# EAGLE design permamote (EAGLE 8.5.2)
AUTHOR: NEAL JACKSON; REV: A; TITLE: MOTE

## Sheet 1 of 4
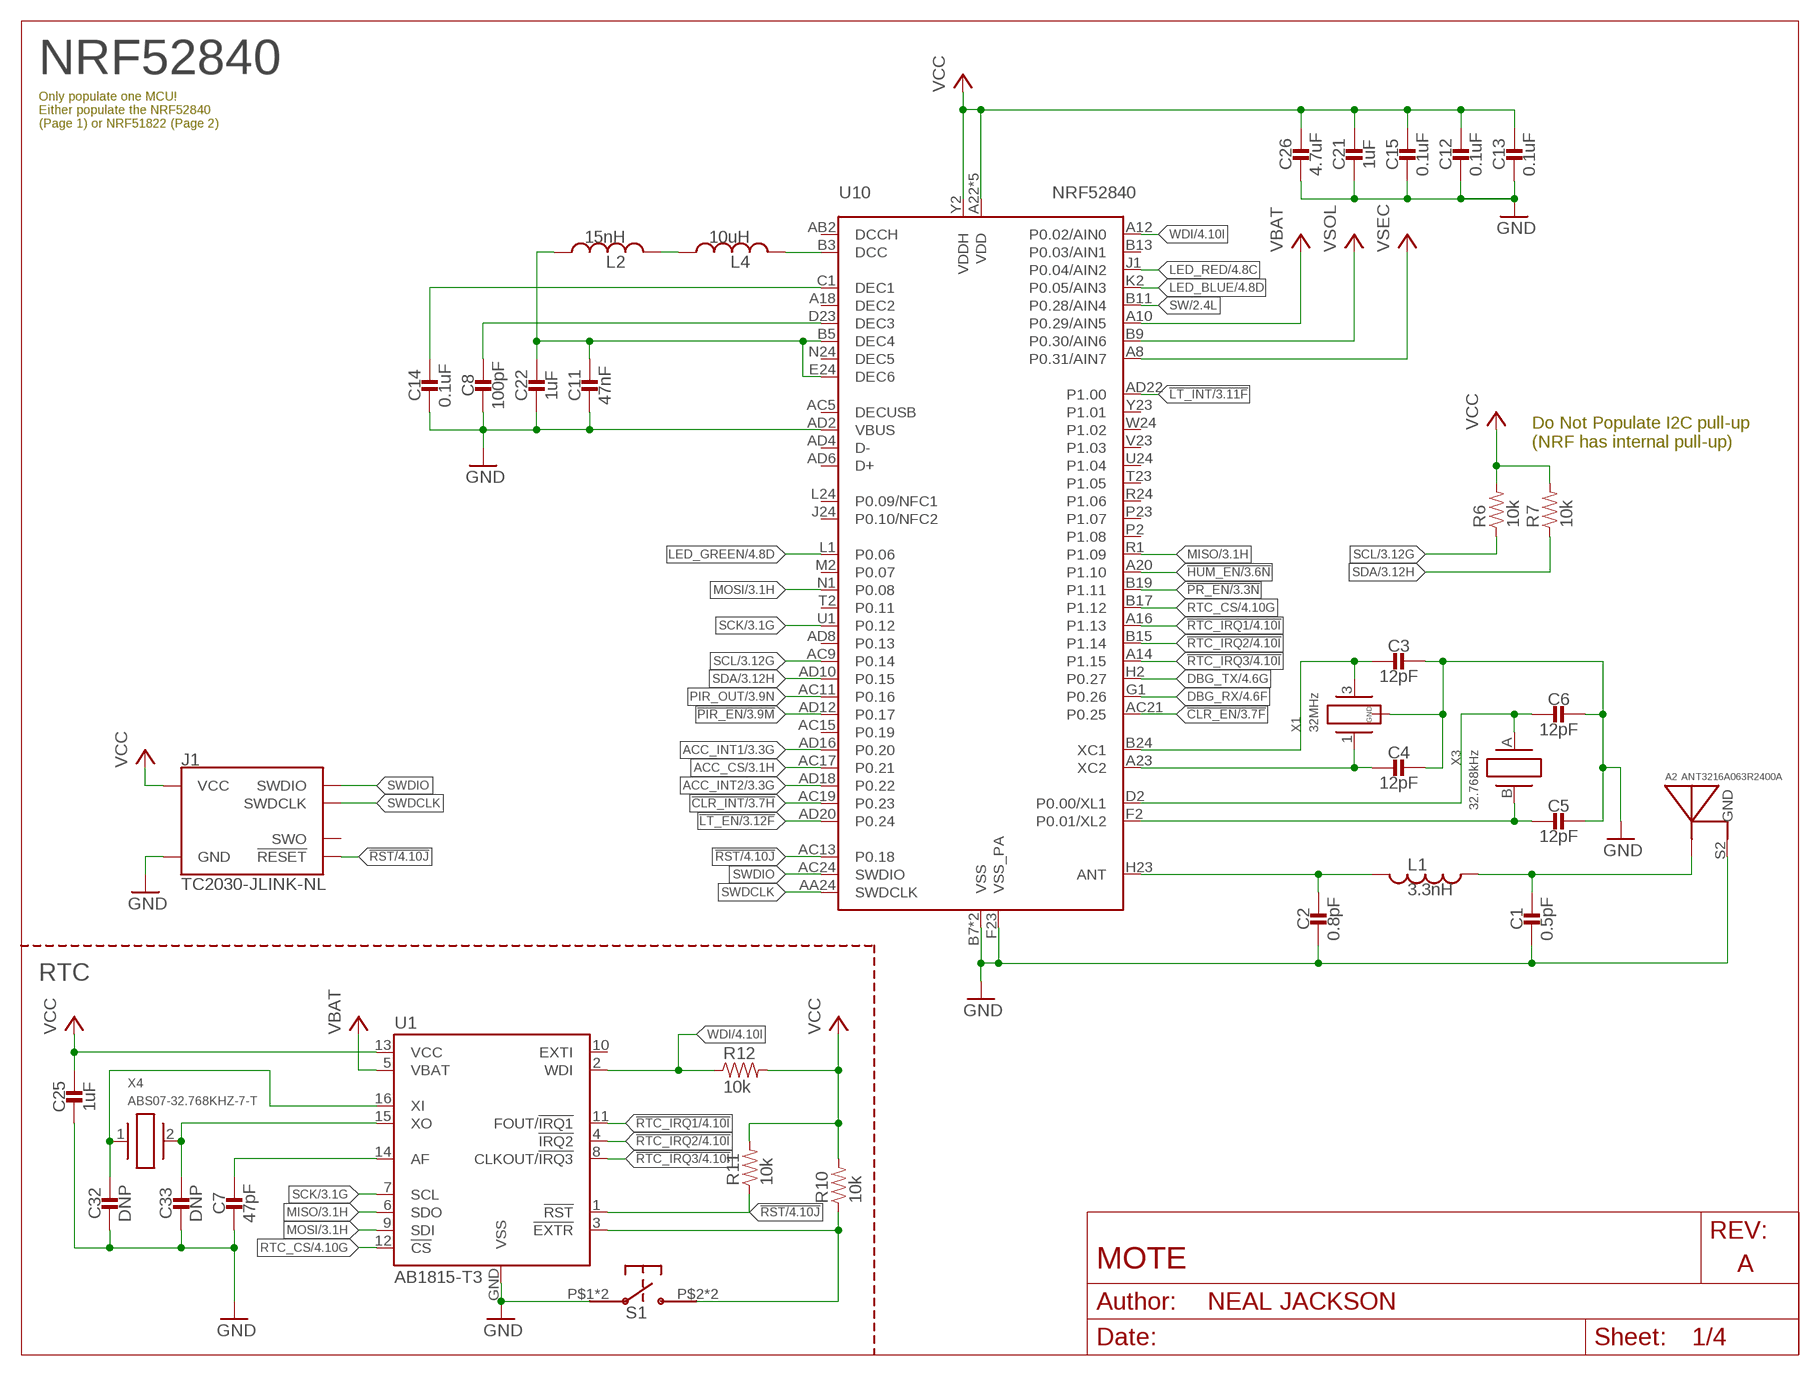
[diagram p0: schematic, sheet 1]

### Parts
A2  ANT3216A063R2400A  [ANT3216A063R2400A]
C1  0.5pF  CAPACITOR0402_CAP  [0402_CAP]
C2  0.8pF  CAPACITOR0402_CAP  [0402_CAP]
C3  12pF  CAPACITOR0402_CAP  [0402_CAP]
C4  12pF  CAPACITOR0402_CAP  [0402_CAP]
C5  12pF  CAPACITOR0402_CAP  [0402_CAP]
C6  12pF  CAPACITOR0402_CAP  [0402_CAP]
C7  47pF  CAPACITOR0402_CAP  [0402_CAP]
C8  100pF  CAPACITOR0402_CAP  [0402_CAP]
C11  47nF  CAPACITOR0402_CAP  [0402_CAP]
C12  0.1uF  CAPACITOR0402_CAP  [0402_CAP]
C13  0.1uF  CAPACITOR0402_CAP  [0402_CAP]
C14  0.1uF  CAPACITOR0402_CAP  [0402_CAP]
C15  0.1uF  CAPACITOR0402_CAP  [0402_CAP]
C21  1uF  CAPACITOR0402_CAP  [0402_CAP]
C22  1uF  CAPACITOR0402_CAP  [0402_CAP]
C25  1uF  CAPACITOR0402_CAP  [0402_CAP]
C26  4.7uF  CAPACITOR0402_CAP  [0402_CAP]
C32  DNP  CAPACITOR0402_CAP  [0402_CAP]
C33  DNP  CAPACITOR0402_CAP  [0402_CAP]
J1  TC2030-JLINK-NL  [TC2030-IDC-NL]
L1  3.3nH  INDUCTOR0402  [0402_CAP]
L2  15nH  INDUCTOR0402  [0402_CAP]
L4  10uH  INDUCTOR0603  [0603_CAP]
R6  10k  RESISTOR0402_RES  [0402_RES]
R7  10k  RESISTOR0402_RES  [0402_RES]
R10  10k  RESISTOR0402_RES  [0402_RES]
R11  10k  RESISTOR0402_RES  [0402_RES]
R12  10k  RESISTOR0402_RES  [0402_RES]
S1  EVQP2  [EVQP2]
U1  AB1815-T3  [QFN-16-3MM]
U10  NRF52840  [AQFN73]
X1  32MHz  7V-32.000MAHV-T  [TXC-7V]
X3  32.768kHz  ABS05-32.768KHZ-9-T  [ABS05]
X4  ABS07-32.768KHZ-7-T  [2-SMD]

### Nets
!CLR_EN: U10.AC21(P0.25) ; also sheet 3,4
!CLR_INT: U10.AC19(P0.23) ; also sheet 3,4
!HUM_EN: U10.A20(P1.10) ; also sheet 3,4
!LT_EN: U10.AD20(P0.24) ; also sheet 3,4
!LT_INT: U10.AD22(P1.00) ; also sheet 3,4
!PIR_EN: U10.AD12(P0.17) ; also sheet 3,4
!PR_EN: U10.B19(P1.11) ; also sheet 3,4
!RST: J1.3(!RESET) R11.1 U1.1(!RST) U10.AC13(P0.18) ; also sheet 4
!RTC_EXTR: R10.1 S1.P$2 S1.P$4 U1.3(!EXTR)
!RTC_IRQ1: U1.11(FOUT/!IRQ1) U10.A16(P1.13) ; also sheet 4
!RTC_IRQ2: U1.4(!IRQ2) U10.B15(P1.14) ; also sheet 4
!RTC_IRQ3: U1.8(CLKOUT/!IRQ3) U10.A14(P1.15) ; also sheet 4
ACC_CS: U10.AC17(P0.21) ; also sheet 3,4
ACC_INT1: U10.AD16(P0.20) ; also sheet 3,4
ACC_INT2: U10.AD18(P0.22) ; also sheet 3,4
DBG_RX: U10.G1(P0.26) ; also sheet 4
DBG_TX: U10.H2(P0.27) ; also sheet 4
GND: A2.S2(GND) C1.2 C2.2 C3.1 C4.1 C5.1 C6.1 C7.2 C8.2 C11.2 C12.2 C13.2 C14.2 C15.2 C21.2 C22.2 C25.2 C26.2 C32.2 C33.2 J1.5(GND) S1.P$1 S1.P$3 U1.GND(VSS) U10.AD2(VBUS) U10.B7(VSS) U10.F23(VSS_PA) U10.GND(VSS) X1.2(GND) X1.4(GND) ; also sheet 2,3,4
LED_BLUE: U10.K2(P0.05/AIN3) ; also sheet 4
LED_GREEN: U10.L1(P0.06) ; also sheet 4
LED_RED: U10.J1(P0.04/AIN2) ; also sheet 4
MISO: U1.6(SDO) U10.R1(P1.09) ; also sheet 3,4
MOSI: U1.9(SDI) U10.N1(P0.08) ; also sheet 3,4
N$2: C14.1 U10.C1(DEC1)
N$3: C11.1 C22.1 L2.1 U10.B5(DEC4) U10.E24(DEC6)
N$4: C8.1 U10.D23(DEC3)
N$5: C2.1 L1.2 U10.H23(ANT)
N$6: A2.S1(ANTENNA) C1.1 L1.1
N$8: C3.2 U10.B24(XC1) X1.3
N$9: C4.2 U10.A23(XC2) X1.1
N$25: C7.1 U1.14(AF)
N$26: C32.1 U1.16(XI) X4.1
N$27: C33.1 U1.15(XO) X4.2
N$44: L4.2 U10.B3(DCC)
N$49: L2.2 L4.1
PIR_OUT: U10.AC11(P0.16) ; also sheet 3,4
RTC_CS: U1.12(!CS) U10.B17(P1.12) ; also sheet 4
SCK: U1.7(SCL) U10.U1(P0.12) ; also sheet 3,4
SCL: R6.1 U10.AC9(P0.14) ; also sheet 3,4
SDA: R7.1 U10.AD10(P0.15) ; also sheet 3,4
SW: U10.B11(P0.28/AIN4) ; also sheet 2,4
SWDCLK: J1.4(SWDCLK) U10.AA24(SWDCLK)
SWDIO: J1.2(SWDIO) U10.AC24(SWDIO)
VBAT: U1.5(VBAT) U10.A10(P0.29/AIN5) ; also sheet 2
VCC: C12.1 C13.1 C15.1 C21.1 C25.1 C26.1 J1.1(VCC) R6.2 R7.2 R10.2 R11.2 R12.2 U1.13(VCC) U10.A22(VDD) U10.AD14(VDD) U10.AD23(VDD) U10.B1(VDD) U10.W1(VDD) U10.Y2(VDDH) ; also sheet 2,3,4
VSEC: U10.A8(P0.31/AIN7) ; also sheet 2,4
VSOL: U10.B9(P0.30/AIN6) ; also sheet 2,4
WDI: R12.1 U1.2(WDI) U10.A12(P0.02/AIN0) ; also sheet 4
XL1: C6.2 U10.D2(P0.00/XL1) X3.A
XL2: C5.2 U10.F2(P0.01/XL2) X3.B
Unconnected: J1.6(SWO) U1.10(EXTI) U10.A18(DEC2) U10.AB2(DCCH) U10.AC5(DECUSB) U10.AC15(P0.19) U10.AD4(D-) U10.AD6(D+) U10.AD8(P0.13) U10.B13(P0.03/AIN1) U10.J24(P0.10/NFC2) U10.L24(P0.09/NFC1) U10.M2(P0.07) U10.N24(DEC5) U10.P2(P1.08) U10.P23(P1.07) U10.R24(P1.06) U10.T2(P0.11) U10.T23(P1.05) U10.U24(P1.04) U10.V23(P1.03) U10.W24(P1.02) U10.Y23(P1.01)

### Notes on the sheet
- NRF52840
- Only populate one MCU!
  Either populate the NRF52840
  (Page 1) or NRF51822 (Page 2)
- Do Not Populate I2C pull-up
  (NRF has internal pull-up)
- RTC

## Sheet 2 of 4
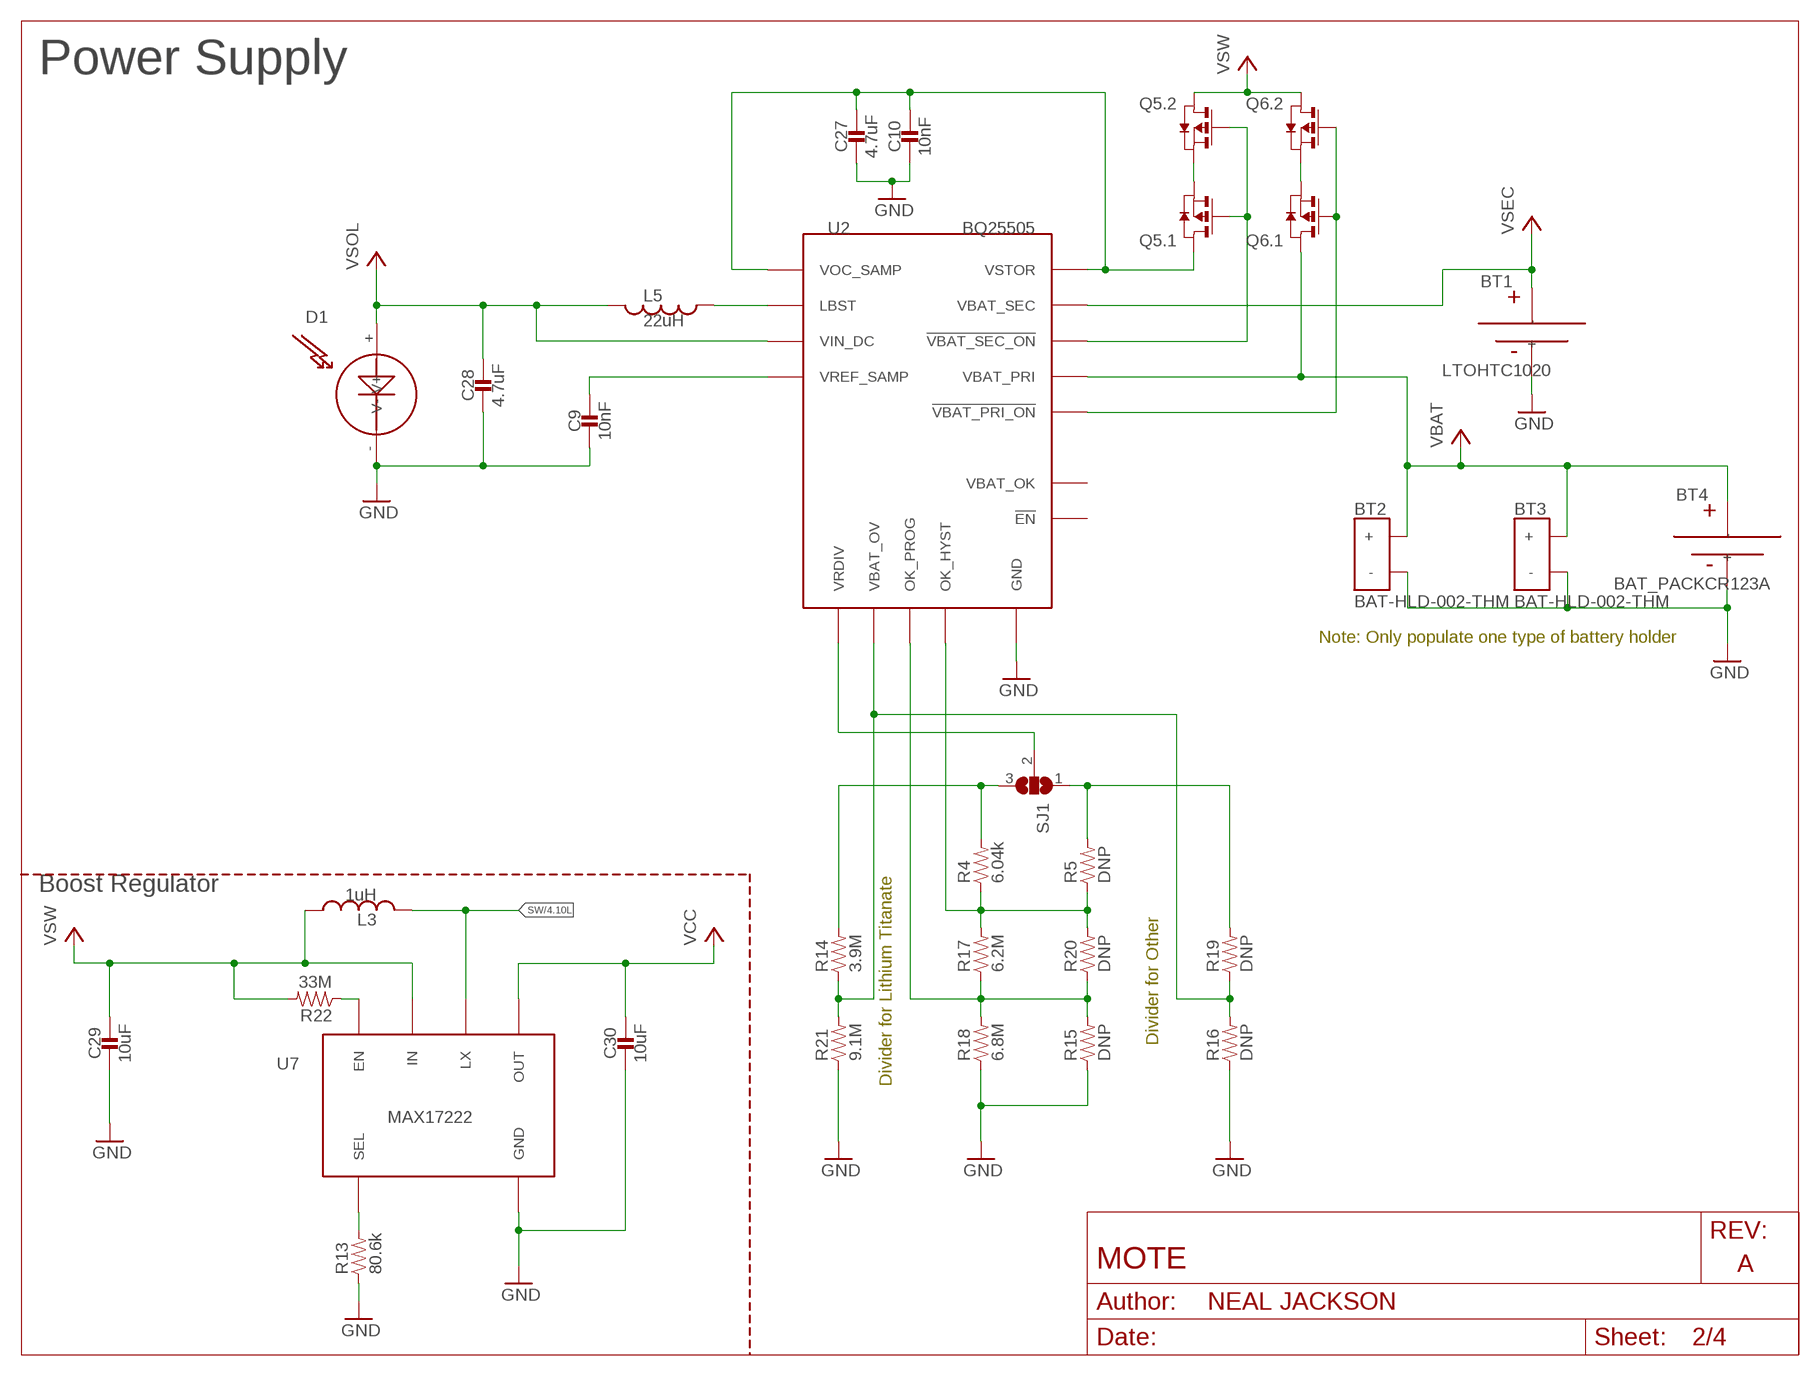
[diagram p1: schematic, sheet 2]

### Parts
BT1  LTOHTC1020  [1020]
BT2  BAT-HLD-002-THM  [BAT-HLD-002-THM]
BT3  BAT-HLD-002-THM  [BAT-HLD-002-THM]
BT4  BAT_PACKCR123A  [BH123A]
C9  10nF  CAPACITOR0402_CAP  [0402_CAP]
C10  10nF  CAPACITOR0402_CAP  [0402_CAP]
C27  4.7uF  CAPACITOR0402_CAP  [0402_CAP]
C28  4.7uF  CAPACITOR0402_CAP  [0402_CAP]
C29  10uF  CAPACITOR0603_CAP  [0603_CAP]
C30  10uF  CAPACITOR0603_CAP  [0603_CAP]
D1  SOLARCELLHOLES  [SOLAR_HOLES]
L3  1uH  INDUCTORIHL  [IHL-1212BZ-11]
L5  22uH  INDUCTOR74437324220  [74437324220]
Q5  PMDXB950UPEL  [XDFN-6]
Q6  PMDXB950UPEL  [XDFN-6]
R4  6.04k  RESISTOR0402_RES  [0402_RES]
R5  DNP  RESISTOR0402_RES  [0402_RES]
R13  80.6k  RESISTOR0603_RES  [0603-RES]
R14  3.9M  RESISTOR0402_RES  [0402_RES]
R15  DNP  RESISTOR0402_RES  [0402_RES]
R16  DNP  RESISTOR0402_RES  [0402_RES]
R17  6.2M  RESISTOR0402_RES  [0402_RES]
R18  6.8M  RESISTOR0402_RES  [0402_RES]
R19  DNP  RESISTOR0402_RES  [0402_RES]
R20  DNP  RESISTOR0402_RES  [0402_RES]
R21  9.1M  RESISTOR0402_RES  [0402_RES]
R22  33M  RESISTOR0603_RES  [0603-RES]
SJ1  SJ2W  [SJ_2]
U2  BQ25505  [S-PVQFN-N20-RGR]
U7  MAX17222  [UDFN-6-MAXIM]

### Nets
!VBAT_PRI_ON: Q6.2(.1:G) Q6.5(.2:G) U2.10(!VBAT_PRI_ON)
!VBAT_SEC_ON: Q5.2(.1:G) Q5.5(.2:G) U2.9(!VBAT_SEC_ON)
GND: BT1.- BT2.GND(-) BT3.GND(-) BT4.- C9.2 C10.2 C27.2 C28.2 C29.2 C30.2 D1.-(V-) R13.1 R15.1 R16.1 R18.1 R21.1 U2.1(GND) U2.6(GND) U2.15(GND) U2.16(GND) U2.17(GND) U2.PAD(GND) U7.3(GND) ; also sheet 1,3,4
LBST: L5.P$1 U2.20(LBST)
N$1: R4.2 R14.2 SJ1.3
N$12: R13.2 U7.4(SEL)
N$14: R22.1 U7.6(EN)
N$16: R5.2 R19.2 SJ1.1
N$18: R14.1 R16.2 R19.1 R21.2 U2.7(VBAT_OV)
N$32: SJ1.2 U2.8(VRDIV)
N$45: Q5.1(.1:S) Q5.4(.2:S)
N$53: Q6.1(.1:S) Q6.4(.2:S)
N$57: R15.2 R17.1 R18.2 R20.1 U2.12(OK_PROG)
N$58: R4.1 R5.1 R17.2 R20.2 U2.11(OK_HYST)
SW: L3.P$2 U7.2(LX) ; also sheet 1,4
VBAT: BT2.POS1(+) BT2.POS2(+) BT2.POS3(+) BT2.POS4(+) BT3.POS1(+) BT3.POS2(+) BT3.POS3(+) BT3.POS4(+) BT4.+ Q6.6(.1:D) U2.14(VBAT_PRI) ; also sheet 1
VCC: C30.1 U7.1(OUT) ; also sheet 1,3,4
VOC_SAMP_VSTOR: C10.1 C27.1 Q5.6(.1:D) U2.3(VOC_SAMP) U2.19(VSTOR)
VREF_SAMP: C9.1 U2.4(VREF_SAMP)
VSEC: BT1.+ U2.18(VBAT_SEC) ; also sheet 1,4
VSOL: C28.1 D1.+(V+) L5.P$2 U2.2(VIN_DC) ; also sheet 1,4
VSW: C29.1 L3.P$1 Q5.3(.2:D) Q6.3(.2:D) R22.2 U7.5(IN)
Unconnected: U2.5(!EN) U2.13(VBAT_OK)

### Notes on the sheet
- Power Supply
- Note: Only populate one type of battery holder
- Boost Regulator
- Divider for Lithium Titanate | Divider for Other

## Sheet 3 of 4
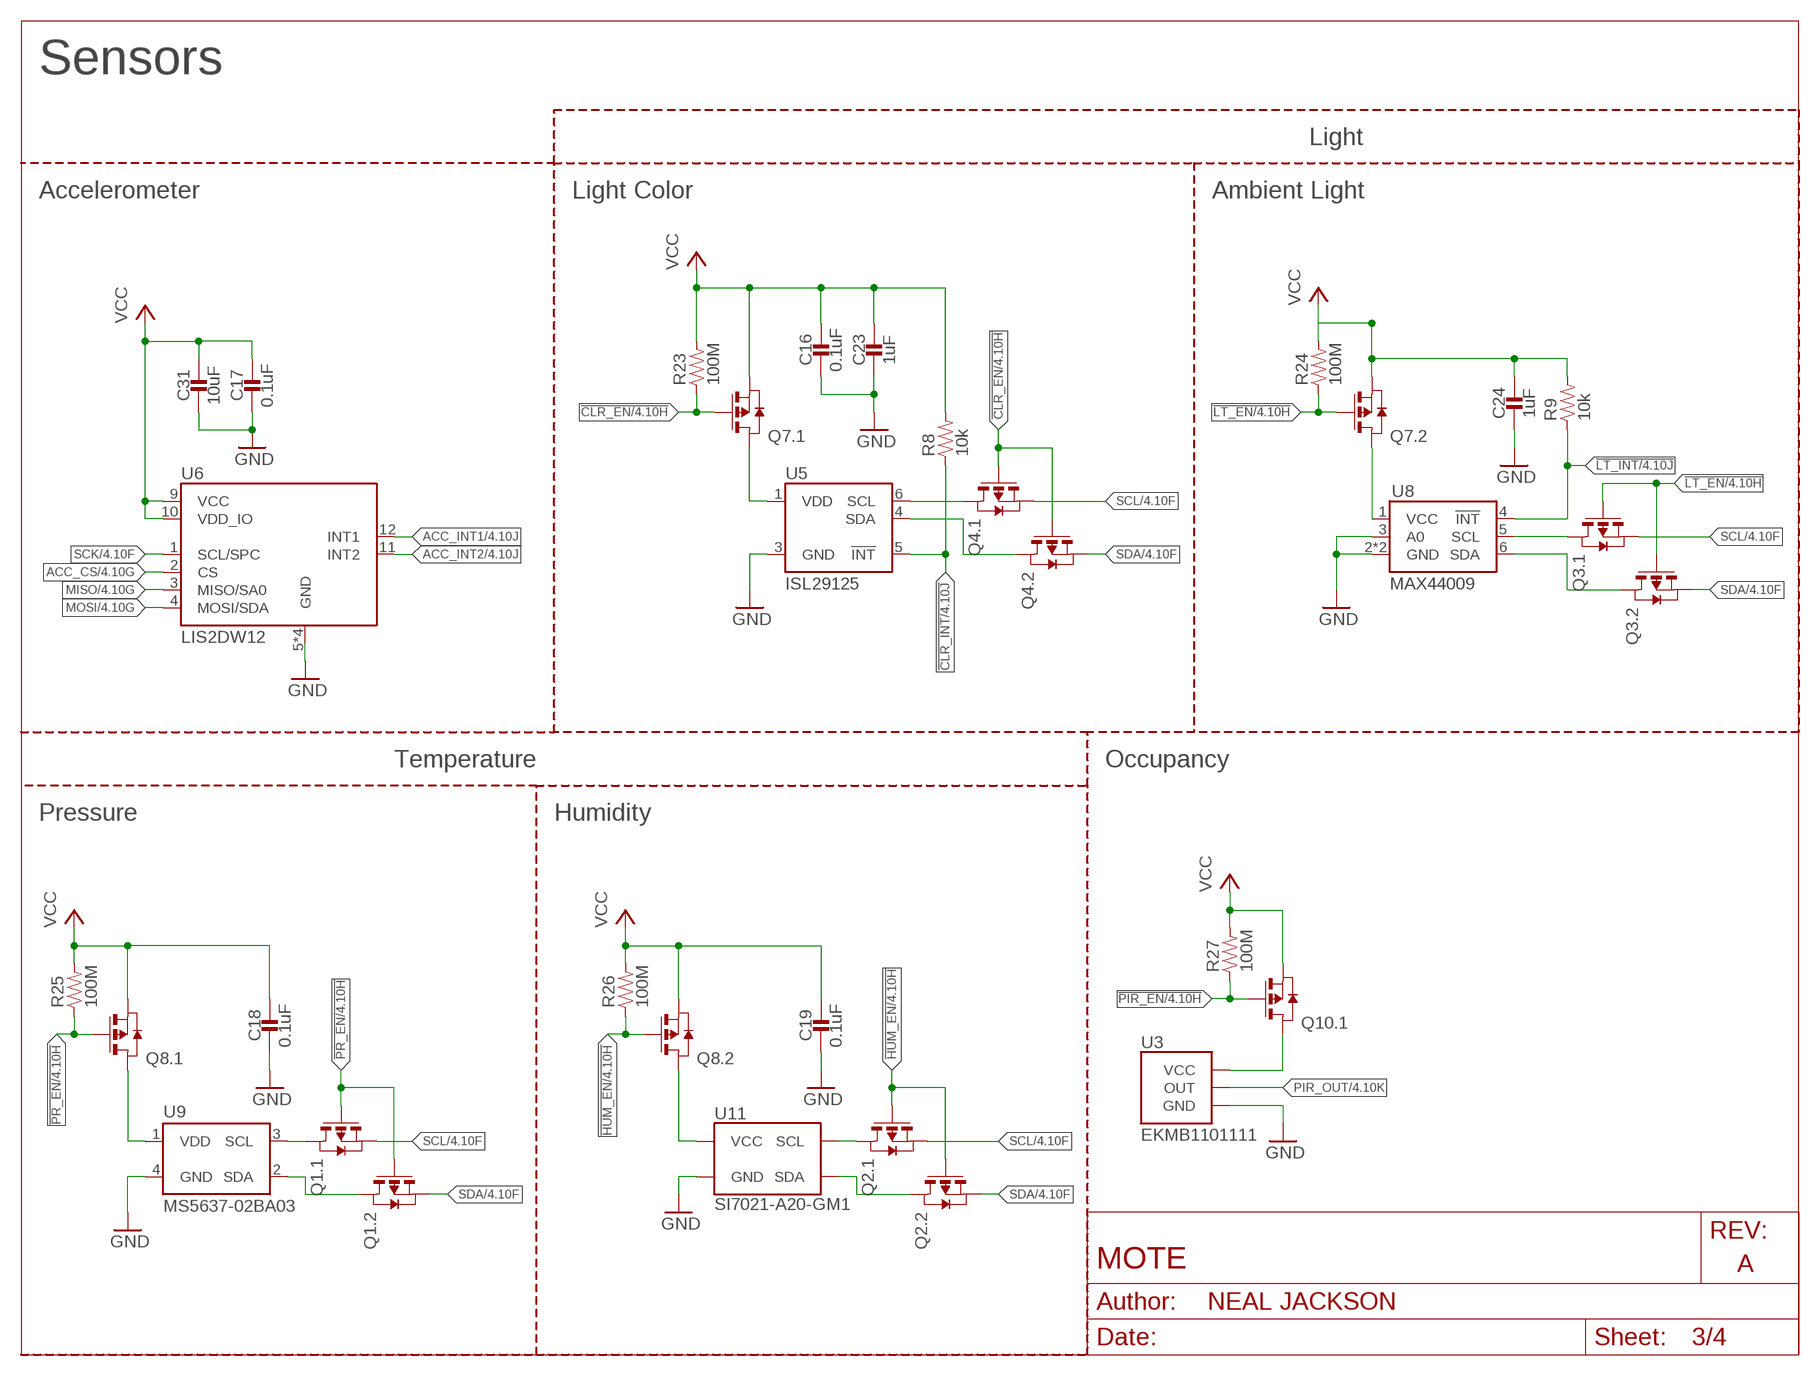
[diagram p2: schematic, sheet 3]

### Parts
C16  0.1uF  CAPACITOR0402_CAP  [0402_CAP]
C17  0.1uF  CAPACITOR0402_CAP  [0402_CAP]
C18  0.1uF  CAPACITOR0402_CAP  [0402_CAP]
C19  0.1uF  CAPACITOR0402_CAP  [0402_CAP]
C23  1uF  CAPACITOR0402_CAP  [0402_CAP]
C24  1uF  CAPACITOR0402_CAP  [0402_CAP]
C31  10uF  CAPACITOR0603_CAP  [0603_CAP]
Q1  PMDXB950UPEL  [XDFN-6]
Q2  PMDXB950UPEL  [XDFN-6]
Q3  PMDXB950UPEL  [XDFN-6]
Q4  PMDXB950UPEL  [XDFN-6]
Q7  PMDXB950UPEL  [XDFN-6]
Q8  PMDXB950UPEL  [XDFN-6]
Q10  PMDXB950UPEL  [XDFN-6]
R8  10k  RESISTOR0402_RES  [0402_RES]
R9  10k  RESISTOR0402_RES  [0402_RES]
R23  100M  RESISTOR0402_RES  [0402_RES]
R24  100M  RESISTOR0402_RES  [0402_RES]
R25  100M  RESISTOR0402_RES  [0402_RES]
R26  100M  RESISTOR0402_RES  [0402_RES]
R27  100M  RESISTOR0402_RES  [0402_RES]
U3  EKMB1101111  [AMN2]
U5  ISL29125  [ODFN-6-1.5MMX1.6MM]
U6  LIS2DW12  [LGA-12]
U8  MAX44009  [UDFN-6-EXPOSED]
U9  MS5637-02BA03  [4-SMD]
U11  SI7021-A20-GM1  [DFN-6/3MM]

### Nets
!CLR_EN: Q4.2(.1:G) Q4.5(.2:G) Q7.2(.1:G) R23.1 ; also sheet 1,4
!CLR_INT: R8.1 U5.5(!INT) ; also sheet 1,4
!HUM_EN: Q2.2(.1:G) Q2.5(.2:G) Q8.5(.2:G) R26.1 ; also sheet 1,4
!LT_EN: Q3.2(.1:G) Q3.5(.2:G) Q7.5(.2:G) R24.1 ; also sheet 1,4
!LT_INT: R9.1 U8.4(!INT) ; also sheet 1,4
!PIR_EN: Q10.2(.1:G) R27.1 ; also sheet 1,4
!PR_EN: Q1.2(.1:G) Q1.5(.2:G) Q8.2(.1:G) R25.1 ; also sheet 1,4
ACC_CS: U6.2(CS) ; also sheet 1,4
ACC_INT1: U6.12(INT1) ; also sheet 1,4
ACC_INT2: U6.11(INT2) ; also sheet 1,4
GND: C16.2 C17.2 C18.2 C19.2 C23.2 C24.2 C31.2 U3.GND U5.3(GND) U6.5(GND) U6.6(GND) U6.7(GND) U6.8(GND) U8.2(GND) U8.3(A0) U8.EP(GND) U9.4(GND) U11.2(GND) ; also sheet 1,2,4
MISO: U6.3(MISO/SA0) ; also sheet 1,4
MOSI: U6.4(MOSI/SDA) ; also sheet 1,4
N$20: Q7.3(.2:D) U8.1(VCC)
N$21: Q8.6(.1:D) U9.1(VDD)
N$22: Q8.3(.2:D) U11.5(VCC)
N$23: Q10.6(.1:D) U3.VCC
N$31: Q7.6(.1:D) U5.1(VDD)
N$34: Q1.6(.1:D) U9.3(SCL)
N$41: Q1.3(.2:D) U9.2(SDA)
N$48: Q2.3(.2:D) U11.1(SDA)
N$50: Q2.6(.1:D) U11.6(SCL)
N$51: Q3.3(.2:D) U8.6(SDA)
N$52: Q3.6(.1:D) U8.5(SCL)
N$54: Q4.3(.2:D) U5.4(SDA)
N$55: Q4.6(.1:D) U5.6(SCL)
PIR_OUT: U3.OUT ; also sheet 1,4
SCK: U6.1(SCL/SPC) ; also sheet 1,4
SCL: Q1.1(.1:S) Q2.1(.1:S) Q3.1(.1:S) Q4.1(.1:S) ; also sheet 1,4
SDA: Q1.4(.2:S) Q2.4(.2:S) Q3.4(.2:S) Q4.4(.2:S) ; also sheet 1,4
VCC: C16.1 C17.1 C18.1 C19.1 C23.1 C24.1 C31.1 Q7.1(.1:S) Q7.4(.2:S) Q8.1(.1:S) Q8.4(.2:S) Q10.1(.1:S) R8.2 R9.2 R23.2 R24.2 R25.2 R26.2 R27.2 U6.9(VCC) U6.10(VDD_IO) ; also sheet 1,2,4
Unconnected: Q10.3(.2:D) Q10.4(.2:S) Q10.5(.2:G)

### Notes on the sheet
- Sensors
- Light
- Accelerometer | Light Color | Ambient Light
- Temperature | Occupancy
- Pressure | Humidity

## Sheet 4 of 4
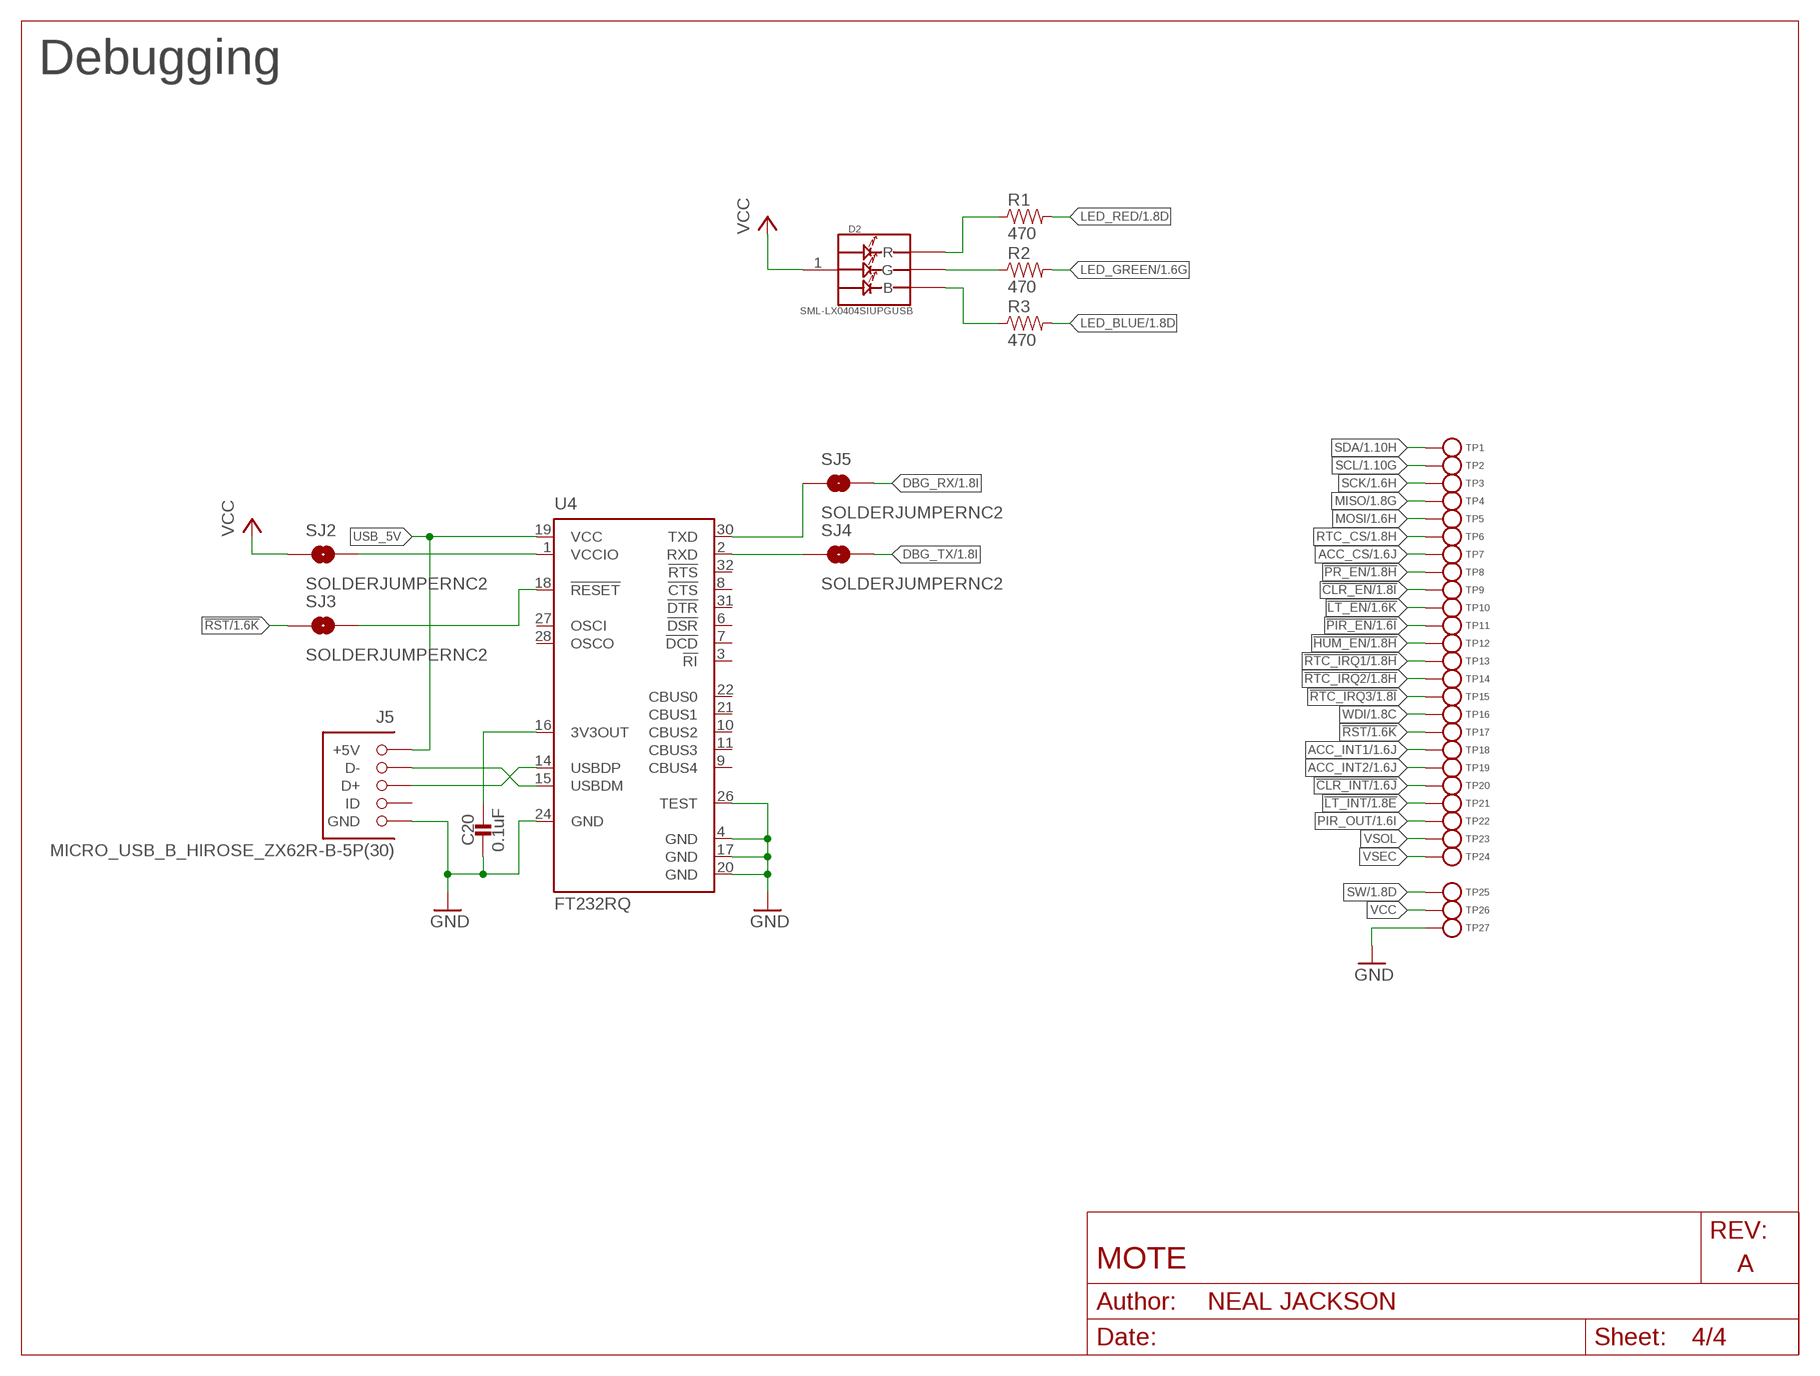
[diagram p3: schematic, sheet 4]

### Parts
C20  0.1uF  CAPACITOR0402_CAP  [0402_CAP]
D2  SML-LX0404SIUPGUSB  [1MM_SQ_4PAD]
J5  MICRO_USB_B_HIROSE_ZX62R-B-5P(30)  [MICRO_USB_B_HIROSE_ZX62R-B-5P(30)]
R1  470  RESISTOR0402_RES  [0402_RES]
R2  470  RESISTOR0402_RES  [0402_RES]
R3  470  RESISTOR0402_RES  [0402_RES]
SJ2  SOLDERJUMPERNC2  [SJ_2S-NOTRACE]
SJ3  SOLDERJUMPERNC2  [SJ_2S-NOTRACE]
SJ4  SOLDERJUMPERNC2  [SJ_2S-NOTRACE]
SJ5  SOLDERJUMPERNC2  [SJ_2S-NOTRACE]
TP1  TEST-POINT  [PAD.03X.03]
TP2  TEST-POINT  [PAD.03X.03]
TP3  TEST-POINT  [PAD.03X.03]
TP4  TEST-POINT  [PAD.03X.03]
TP5  TEST-POINT  [PAD.03X.03]
TP6  TEST-POINT  [PAD.03X.03]
TP7  TEST-POINT  [PAD.03X.03]
TP8  TEST-POINT  [PAD.03X.03]
TP9  TEST-POINT  [PAD.03X.03]
TP10  TEST-POINT  [PAD.03X.03]
TP11  TEST-POINT  [PAD.03X.03]
TP12  TEST-POINT  [PAD.03X.03]
TP13  TEST-POINT  [PAD.03X.03]
TP14  TEST-POINT  [PAD.03X.03]
TP15  TEST-POINT  [PAD.03X.03]
TP16  TEST-POINT  [PAD.03X.03]
TP17  TEST-POINT  [PAD.03X.03]
TP18  TEST-POINT  [PAD.03X.03]
TP19  TEST-POINT  [PAD.03X.03]
TP20  TEST-POINT  [PAD.03X.03]
TP21  TEST-POINT  [PAD.03X.03]
TP22  TEST-POINT  [PAD.03X.03]
TP23  TEST-POINT  [PAD.03X.03]
TP24  TEST-POINT  [PAD.03X.03]
TP25  TEST-POINT  [PAD.03X.03]
TP26  TEST-POINT  [PAD.03X.03]
TP27  TEST-POINT  [PAD.03X.03]
U4  FT232RQ  [QFN32]

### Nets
!CLR_EN: TP9.P$1(TESTPOINT) ; also sheet 1,3
!CLR_INT: TP20.P$1(TESTPOINT) ; also sheet 1,3
!FTDI_RESET: SJ3.2 U4.18(!RESET)
!HUM_EN: TP12.P$1(TESTPOINT) ; also sheet 1,3
!LT_EN: TP10.P$1(TESTPOINT) ; also sheet 1,3
!LT_INT: TP21.P$1(TESTPOINT) ; also sheet 1,3
!PIR_EN: TP11.P$1(TESTPOINT) ; also sheet 1,3
!PR_EN: TP8.P$1(TESTPOINT) ; also sheet 1,3
!RST: SJ3.1 TP17.P$1(TESTPOINT) ; also sheet 1
!RTC_IRQ1: TP13.P$1(TESTPOINT) ; also sheet 1
!RTC_IRQ2: TP14.P$1(TESTPOINT) ; also sheet 1
!RTC_IRQ3: TP15.P$1(TESTPOINT) ; also sheet 1
ACC_CS: TP7.P$1(TESTPOINT) ; also sheet 1,3
ACC_INT1: TP18.P$1(TESTPOINT) ; also sheet 1,3
ACC_INT2: TP19.P$1(TESTPOINT) ; also sheet 1,3
D+: J5.3(D+) U4.14(USBDP)
D-: J5.2(D-) U4.15(USBDM)
DBG_RX: SJ5.2 ; also sheet 1
DBG_TX: SJ4.2 ; also sheet 1
FTDI_VCCIO: SJ2.2 U4.1(VCCIO)
GND: C20.2 J5.5(GND) TP27.P$1(TESTPOINT) U4.4(GND) U4.17(GND) U4.20(GND) U4.24(GND) U4.26(TEST) ; also sheet 1,2,3
LED_BLUE: R3.2 ; also sheet 1
LED_GREEN: R2.2 ; also sheet 1
LED_RED: R1.2 ; also sheet 1
MISO: TP4.P$1(TESTPOINT) ; also sheet 1,3
MOSI: TP5.P$1(TESTPOINT) ; also sheet 1,3
N$13: C20.1 U4.16(3V3OUT)
N$15: D2.2(R) R1.1
N$17: D2.4(G) R2.1
N$19: D2.3(B) R3.1
PIR_OUT: TP22.P$1(TESTPOINT) ; also sheet 1,3
RTC_CS: TP6.P$1(TESTPOINT) ; also sheet 1
RXD: SJ4.1 U4.2(RXD)
SCK: TP3.P$1(TESTPOINT) ; also sheet 1,3
SCL: TP2.P$1(TESTPOINT) ; also sheet 1,3
SDA: TP1.P$1(TESTPOINT) ; also sheet 1,3
SW: TP25.P$1(TESTPOINT) ; also sheet 1,2
TXD: SJ5.1 U4.30(TXD)
USB_5V: J5.1(+5V) U4.19(VCC)
VCC: D2.1(VDD) SJ2.1 TP26.P$1(TESTPOINT) ; also sheet 1,2,3
VSEC: TP24.P$1(TESTPOINT) ; also sheet 1,2
VSOL: TP23.P$1(TESTPOINT) ; also sheet 1,2
WDI: TP16.P$1(TESTPOINT) ; also sheet 1
Unconnected: J5.4(ID) U4.3(!RI) U4.6(!DSR) U4.7(!DCD) U4.8(!CTS) U4.9(CBUS4) U4.10(CBUS2) U4.11(CBUS3) U4.21(CBUS1) U4.22(CBUS0) U4.27(OSCI) U4.28(OSCO) U4.31(!DTR) U4.32(!RTS)

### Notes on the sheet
- Debugging

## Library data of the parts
A2 = chips:ANT3216A063R2400A: Yageo 2.4GHz; DIGIKEY: 311-1542-1-ND; MANUFACTURER: YAGEO; MPN: ANT3216A063R2400A
BT1 = batteries:LTOHTC
BT2 BT3 = batteries:BAT-HLD-002-THM: RETAINER BATT CR2016 PC PINS; DIGIKEY: BAT-HLD-001-THM-ND; MOUSER: 712-BAT-HLD-001-THM; MPN: BAT-HLD-001-THM
BT4 = batteries:BAT_PACK: collection of battery footprints; DIGIKEY: BH123A-ND; MANUFACTURER: MPD; MPN: BH123A
C1 = passives:CAPACITOR: SMD Capacitor; DIGIKEY: 490-6264-1-ND; MPN: GRM1555C1HR50WA01D
C2 = passives:CAPACITOR: SMD Capacitor; DIGIKEY: 490-6269-1-ND; MPN: GRM1555C1HR80BA01D
C3-C6 = passives:CAPACITOR: SMD Capacitor; DIGIKEY: 490-6197-1-ND; MPN: GRM1555C1H120GA01D
C7 = passives:CAPACITOR: SMD Capacitor; DIGIKEY: 490-5942-1-ND; MPN: GRM1555C1H470JA01D
C8 = passives:CAPACITOR: SMD Capacitor; DIGIKEY: 490-5922-1-ND; MPN: GRM1555C1H101JA01D
C9 C10 = passives:CAPACITOR: SMD Capacitor; DIGIKEY: 490-4516-1-ND; MPN: GRM155R71H103KA88D
C11 = passives:CAPACITOR: SMD Capacitor; DIGIKEY: 445-1264-1-ND; MPN: C1005X7R1C473K050BC
C12-C20 = passives:CAPACITOR: SMD Capacitor; DIGIKEY: 490-6328-1-ND; MPN: GRM155R71C104KA88J
C21-C25 = passives:CAPACITOR: SMD Capacitor; DIGIKEY: 490-7195-1-ND; MPN: GRM155R70G105KA12D
C26-C28 = passives:CAPACITOR: SMD Capacitor; DIGIKEY: 445-5947-1-ND; MPN: C1005X5R0J475K050BC
C29-C31 = passives:CAPACITOR: SMD Capacitor; DIGIKEY: 490-3896-1-ND; MPN: GRM188R60J106ME47D
C32 C33 = passives:CAPACITOR: SMD Capacitor
D1 = permamote:SOLARCELL: Generic solar cell
D2 = leds:SML-LX0404SIUPGUSB: 1mm^2 RGB LED; DIGIKEY: 67-2125-1-ND; MANUFACTURER: Lumex Opto; MPN: SML-LX0404SIUPGUSB
J1 = connector:TC2030-JLINK
J5 = connector:MICRO_USB_B_HIROSE_ZX62R-B-5P(30): USB Micro B Connector Rounded side is up.; DIGIKEY: H125274CT-ND; MOUSER: 798-ZX62R-B-5P30; MPN: ZX62R-B-5P(30); NEWARK: 84Y6712
L1 = passives:INDUCTOR: A very specific inductor; DIGIKEY: 535-10426-1-ND; MPN: AISC-0402-3N3J-T
L2 = passives:INDUCTOR: A very specific inductor; DIGIKEY: 587-1521-1-ND; MPN: HK100515NJ-T
L3 = passives:INDUCTOR: A very specific inductor; DIGIKEY: 541-1319-1-ND; MANUFACTURER: Vishay Dale; MPN: IHLP1212BZER1R0M11
L4 = passives:INDUCTOR: A very specific inductor; DIGIKEY: 490-4025-1-ND; MPN: LQM18FN100M00D
L5 = passives:INDUCTOR: A very specific inductor; DIGIKEY: 732-3340-1-ND; MPN: 74437324220
Q1-Q8 Q10 = fets:PMDXB950UPEL: 20 V 500mA, dual P-channel Trench MOSFET; DIGIKEY: 1727-2601-1-ND; MANUFACTURER: NEXPERIA; MPN: PMDXB950UPELZ
R1-R3 = passives:RESISTOR: Resistor; DIGIKEY: 311-470JRCT-ND; MPN: RC0402JR-07470RL
R4 = passives:RESISTOR: Resistor; DIGIKEY: YAG2293CT-ND; MPN: RC0402FR-076K04L
R5 R15 R16 R19 R20 = passives:RESISTOR: Resistor; DIGIKEY: YAG3306CT-ND
R6-R12 = passives:RESISTOR: Resistor; DIGIKEY: 311-10KJRCT-ND; MPN: RC0402JR-0710KL
R13 = passives:RESISTOR: Resistor; DIGIKEY: 311-80.6KHRCT-ND; MPN: RC0603FR-0780K6L
R14 = passives:RESISTOR: Resistor; DIGIKEY: YAG3301CT-ND; MPN: RC0402JR-073M9L
R17 = passives:RESISTOR: Resistor; DIGIKEY: YAG3309CT-ND; MPN: RC0402JR-076M2L
R18 = passives:RESISTOR: Resistor; DIGIKEY: YAG3310CT-ND; MPN: RC0402JR-076M8L
R21 = passives:RESISTOR: Resistor; DIGIKEY: YAG3322CT-ND; MPN: RC0402JR-079M1L
R22 = passives:RESISTOR: Resistor; DIGIKEY: HMC0603JT33M0CT-ND; MPN: HMC0603JT33M0
R23-R27 = passives:RESISTOR: Resistor; DIGIKEY: 541-100MAHCT-ND; MPN: HMC0402JT100M
S1 = switches:EVQP2: SWITCH TACTILE SPST-NO 0.02A 15V; DIGIKEY: P11084SCT-ND; MPN: EVQ-P2K02Q
SJ1 = jumper:SJ2W: SMD solder JUMPER
SJ2-SJ5 = SparkFun-Passives:SOLDERJUMPER: Solder Jumper
TP1-TP27 = headers:TEST-POINT
U1 = chips:AB1815-T3: Ultra-low current RTC. 55nA quiescent @ 3V. 1.5-3.6V input.; DIGIKEY: 535-11936-1-ND; MANUFACTURER: Abracon; MPN: AB1815-T3
U2 = chips:BQ25505: EH front end for switching between primary and secondary cells; DIGIKEY: 296-37078-1-ND; MANUFACTURER: TI; MPN: BQ25505RGRR
U3 = chips:EKMB: Passive infrared human detection sensor with built-in amp.; DIGIKEY: 255-3065-ND; MANUFACTURER: PANASONIC; MPN: EKMB1101111
U4 = ftdichip:FT232R: Source: http://www.ftdichip.com/Documents/DataSheets/DS_FT232R_v104.pdf; MPN: FT232RQ; OC_FARNELL: 1146033; OC_NEWARK: 91K9919
U5 = chips:ISL29125: low power i2c color sensor; DIGIKEY: ISL29125IROZ-T7ACT-ND; MANUFACTURER: INTERSIL; MPN: ISL29125IROZ-T7A
U6 = chips:LIS2DW12: ultra low power 3 axis accelerometer; MANUFACTURER: STMicroelectronics; MOUSER: 511-LIS2DW12TR; MPN: LIS2DW12TR
U7 = chips:MAX17222: Very high efficiency, very low power boost converter suitable for EH applications; DIGIKEY: MAX17222ELT+TCT-ND; MANUFACTURER: MAXIM INTEGRATED; MPN: MAX17222ELT+T
U8 = chips:MAX44009: low power ambient light sensor; DIGIKEY: MAX44009EDT+TCT-ND; MANUFACTURER: MAXIM; MPN: MAX44009EDT+T
U9 = chips:MS5637-02BA03: low power pressure sensor; DIGIKEY: 223-1199-1-ND; MANUFACTURER: TE CONNECTIVITY; MPN: MS563702BA03-50
U10 = chips:NRF52840: ultra-low power 2.4 GHz wireless system on chip (SoC) integrating a multiprotocol 2.4 GHz transceiver, an ARM® Cortex®-M4F CPU.; DIGIKEY: 1490-1071-1-ND; MANUFACTURER: NORIDIC SEMICONDUCTOR; MPN: NRF52840
U11 = chips:SI7021: IC TEMP SENSOR RH 2% DFN; DIGIKEY: 336-3141-ND; MOUSER: 634-SI7021-A20-GM1; MPN: SI7021-A20-GM1
X1 = crystals:7V: TXC CRYSTAL SMD; DIGIKEY: 887-2568-1-ND; MANUFACTURER: TXC CORPORATION; MPN: 7M-32.000MAHV-T
X3 = crystals:ABS05-32.768KHZ: 32.768kHz Crystal; DIGIKEY: 535-11897-1-ND; MANUFACTURER: Abracon; MPN: ABS05-32.768KHZ-9-T
X4 = crystals:ABS07-32.768KHZ: 32.768kHz Crystal; DIGIKEY: 535-9543-1-ND; MANUFACTURER: ABRACON; MPN: ABS07-32.768KHZ-7-T

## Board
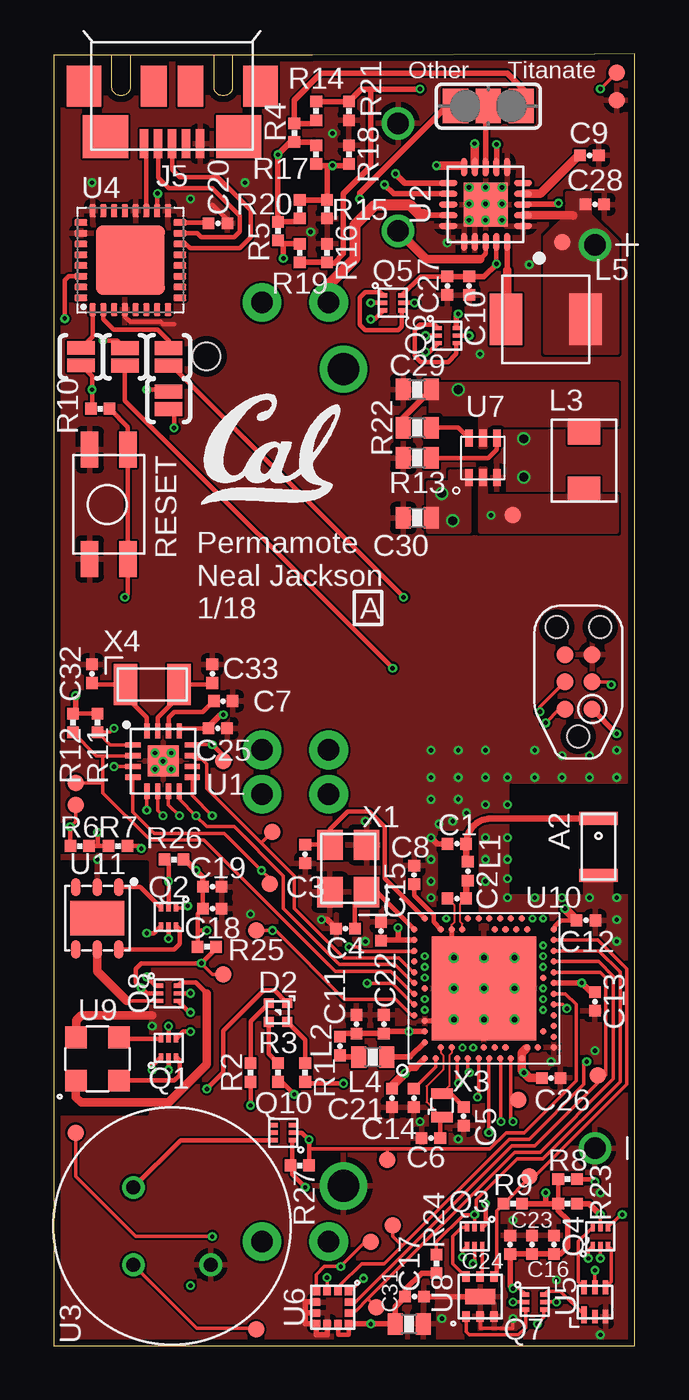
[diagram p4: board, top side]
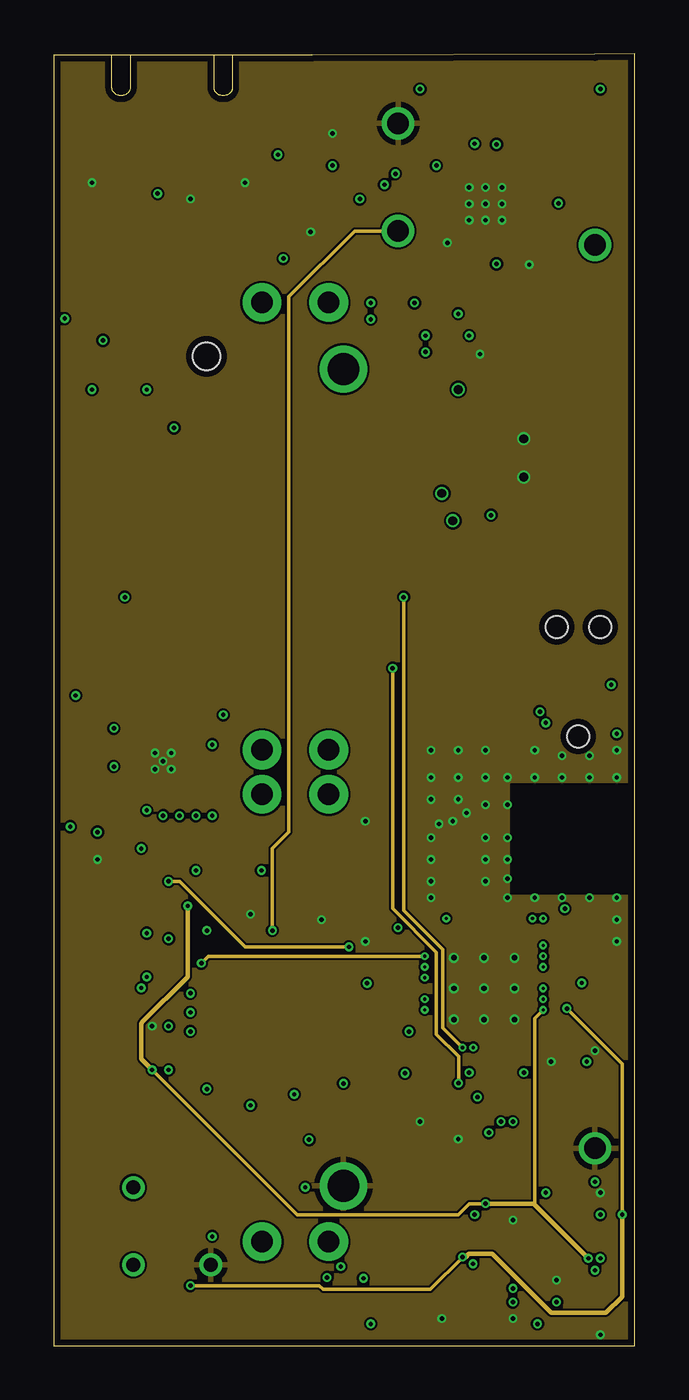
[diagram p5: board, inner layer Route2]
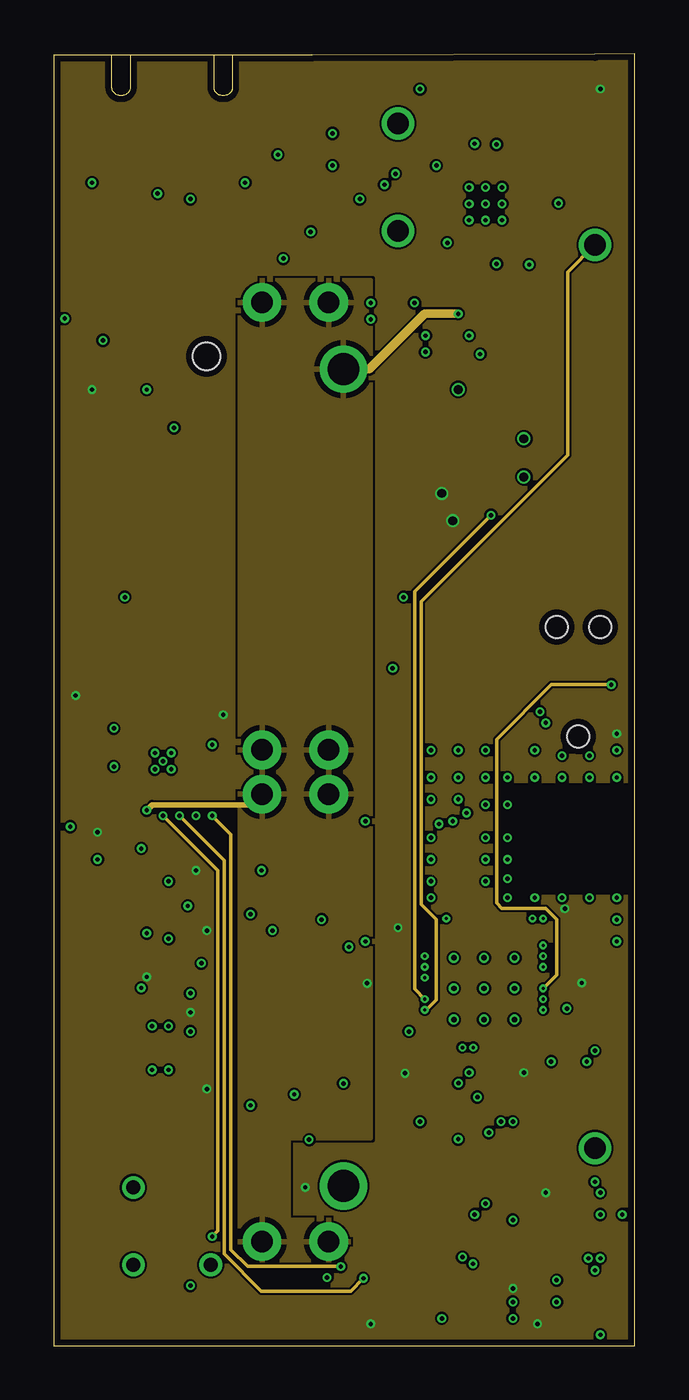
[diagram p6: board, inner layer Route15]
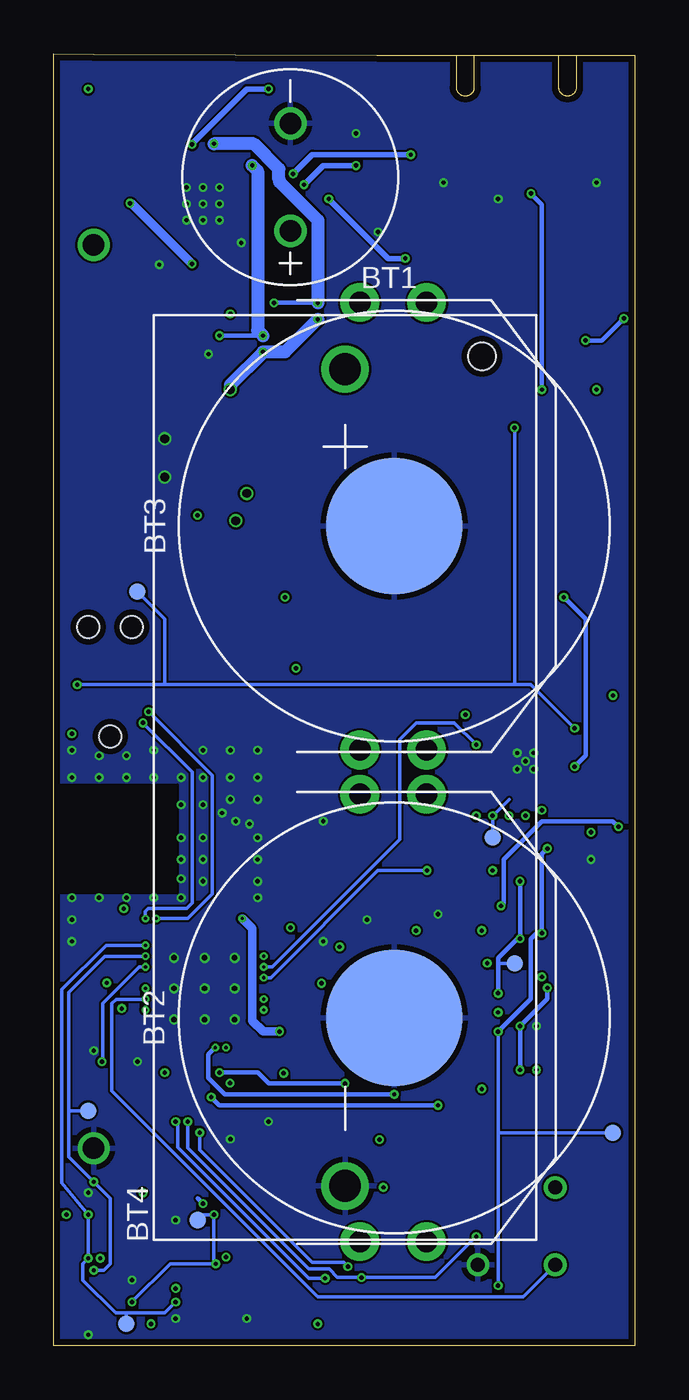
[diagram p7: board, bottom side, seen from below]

Size 27 x 60.06 mm. Coordinates in mm from the lower left corner, seen from the top.
Outline: 0,0 27,0 27,60.06 25.15,60.04 12,60 0,60 0,0
Copper layers (1+2*15+16): Top 0.0178mm / dielectric 59mil / Route2 0.0356mm / dielectric 0.1499mm / Route15 0.0356mm / dielectric 0.2007mm / Bottom 0.0178mm
Design rules "quickturn_co_kr_1oz_4lyr *": minimum track width 4mil, minimum drill 8mil, track to track 4mil, track to pad 4mil, pad to pad 4mil, via to via 4mil, smd to smd 4mil, copper to edge 12mil, drill to drill 12mil, minimum pad ring 8mil, minimum via ring 4mil, stop-mask expansion 3mil, vias tented up to drill 50mil, thermal gap 10mil
tKeepout: area 13.4,0.8 to 13.5,1.3
tRestrict: area 11.9,1.8 to 12.4,1.8; area 11.9,1.3 to 12.4,1.3; area 12.4,0.8 to 12.5,1.3; area 20.1,1.1 to 20.2,1.7

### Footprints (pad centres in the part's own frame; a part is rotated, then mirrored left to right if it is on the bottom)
ANT3216A063R2400A = smd 0.6 x 1.8: S1 -1.325,0; S2 1.325,0
1020 = drill 1: + -2.5,0; - 2.5,0
BAT-HLD-002-THM = smd 6.35 x 6.35: GND 0,0 | drill 1 pad 1.8: POS1 -10.4,1.5; POS2 -10.4,-1.6; POS3 10.4,1.5; POS4 10.4,-1.6
BH123A = drill 1.47: + 18.985,0; - -18.985,0 | hole 1.27: 19.58,-6.37
0402_CAP = smd 0.536 x 0.546: 1 -0.433,0; 2 0.433,0
0603_CAP = smd 0.7 x 1: 1 -0.65,0; 2 0.65,0
SOLAR_HOLES = drill 1: + 0,0; - 42,0
1MM_SQ_4PAD = smd 0.457 x 0.457: 1 0.432,0.432; 2 0.432,-0.432; 3 -0.432,-0.432; 4 -0.432,0.432
TC2030-IDC-NL = smd 0.787 x 0.787: 1 -1.27,-0.635; 2 -1.27,0.635; 3 0,-0.635; 4 0,0.635; 5 1.27,-0.635; 6 1.27,0.635 | hole 1.016: -2.54,0; 2.54,1.016; 2.54,-1.016
MICRO_USB_B_HIROSE_ZX62R-B-5P(30) = smd 0.4 x 1.35: 1 1.3,4.125; 2 0.65,4.125; 3 0,4.125; 4 -0.65,4.125; 5 -1.3,4.125 | smd 2.1 x 2: P$1 3.1,3.8; P$2 -3.1,3.8 | smd 1.6 x 1.9: P$3 -4.1,1.45; P$6 4.1,1.45 | smd 1.2 x 1.9: P$4 -0.85,1.45; P$5 0.85,1.45
IHL-1212BZ-11 = smd 1.2 x 1.5: P$1 -1.35,0; P$2 1.35,0
74437324220 = smd 1.5 x 2.4: P$1 1.85,0; P$2 -1.85,0
XDFN-6 = smd 0.35 x 0.2: 1 -0.425,0.35; 2 -0.425,0; 3 -0.425,-0.35; 4 0.425,-0.35; 5 0.425,0; 6 0.425,0.35
0402_RES = smd 0.536 x 0.546: 1 -0.433,0; 2 0.433,0
0603-RES = smd 0.7 x 1: 1 -0.65,0; 2 0.65,0
EVQP2 = smd 1.676 x 0.813: P$1 -2.54,-0.87; P$2 -2.54,0.908; P$3 2.54,-0.87; P$4 2.54,0.908
SJ_2 = smd 1.168 x 1.6: 1 -1.524,0; 2 0,0; 3 1.524,0
SJ_2S-NOTRACE = smd 0.635 x 1.27: 1 -0.401,0; 2 0.413,0
PAD.03X.03 = smd 0.762 x 0.762: P$1 0,0
QFN-16-3MM = smd 0.7 x 0.25: 1 -1.4,0.75; 2 -1.4,0.25; 3 -1.4,-0.25; 4 -1.4,-0.75; 9 1.35,-0.75; 10 1.35,-0.25; 11 1.35,0.25; 12 1.35,0.75 | smd 0.25 x 0.7: 5 -0.75,-1.4; 6 -0.25,-1.4; 7 0.25,-1.4; 8 0.75,-1.4; 13 0.75,1.4; 14 0.25,1.4; 15 -0.25,1.4; 16 -0.75,1.4 | smd 1.45 x 1.45: GND 0,0
S-PVQFN-N20-RGR = smd 0.28 x 0.85: 1 -1,-1.74; 2 -0.5,-1.74; 3 0,-1.74; 4 0.5,-1.74; 5 1,-1.74; 11 1,1.74; 12 0.5,1.74; 13 0,1.74; 14 -0.5,1.74; 15 -1,1.74 | smd 0.85 x 0.28: 6 1.74,-1; 7 1.74,-0.5; 8 1.74,0; 9 1.74,0.5; 10 1.74,1; 16 -1.74,1; 17 -1.74,0.5; 18 -1.74,0; 19 -1.74,-0.5; 20 -1.74,-1 | smd 2.05 x 2.05: PAD 0,0
AMN2 = drill 0.65: GND 1.796,-1.796; OUT -1.796,-1.796; VCC -1.796,1.796
QFN32 = smd 0.6 x 0.3: 1 -2.3,1.75; 2 -2.3,1.25; 3 -2.3,0.75; 4 -2.3,0.25; 5 -2.3,-0.25; 6 -2.3,-0.75; 7 -2.3,-1.25; 8 -2.3,-1.75; 17 2.3,-1.75; 18 2.3,-1.25; 19 2.3,-0.75; 20 2.3,-0.25; 21 2.3,0.25; 22 2.3,0.75; 23 2.3,1.25; 24 2.3,1.75 | smd 0.3 x 0.6: 9 -1.75,-2.3; 10 -1.25,-2.3; 11 -0.75,-2.3; 12 -0.25,-2.3; 13 0.25,-2.3; 14 0.75,-2.3; 15 1.25,-2.3; 16 1.75,-2.3; 25 1.75,2.3; 26 1.25,2.3; 27 0.75,2.3; 28 0.25,2.3; 29 -0.25,2.3; 30 -0.75,2.3; 31 -1.25,2.3; 32 -1.75,2.3 | smd 3.2 x 3.2: EXP 0,0
ODFN-6-1.5MMX1.6MM = smd 0.8 x 0.25: 1 -0.6,0.5 | smd 0.65 x 0.25: 2 -0.675,0; 3 -0.675,-0.5; 4 0.675,-0.5; 5 0.675,0; 6 0.675,0.5
LGA-12 = smd 0.375 x 0.35: 1 -0.75,0.75; 2 -0.75,0.25; 3 -0.75,-0.25; 4 -0.75,-0.75; 7 0.75,-0.75; 8 0.75,-0.25; 9 0.75,0.25; 10 0.75,0.75 | smd 0.35 x 0.375: 5 -0.25,-0.75; 6 0.25,-0.75; 11 0.25,0.75; 12 -0.25,0.75
UDFN-6-MAXIM = smd 0.8 x 0.35: 1 -0.915,0.65; 2 -0.915,0; 3 -0.915,-0.65; 4 0.915,-0.65; 5 0.915,0; 6 0.915,0.65
UDFN-6-EXPOSED = smd 0.48 x 0.36: 1 -0.925,0.65; 2 -0.925,0; 3 -0.925,-0.65; 4 0.925,-0.65; 5 0.925,0; 6 0.925,0.65 | smd 0.71 x 1.4: EP 0,0
4-SMD = smd 1 x 1: 1 -1,1; 2 -1,-1; 3 1,-1; 4 1,1
AQFN73 = smd 0.3 x 0.3: A8 -1.25,3.25; A10 -0.75,3.25; A12 -0.25,3.25; A14 0.25,3.25; A16 0.75,3.25; A18 1.25,3.25; A20 1.75,3.25; A22 2.25,3.25; A23 2.75,3.25; AA24 3.25,-2.25; AB2 -2.75,-2.5; AC5 -2,-2.75; AC9 -1,-2.75; AC11 -0.5,-2.75; AC13 0,-2.75; AC15 0.5,-2.75; AC17 1,-2.75; AC19 1.5,-2.75; AC21 2,-2.75; AC24 3.25,-2.75; AD2 -2.75,-3.25; AD4 -2.25,-3.25; AD6 -1.75,-3.25; AD8 -1.25,-3.25; AD10 -0.75,-3.25; AD12 -0.25,-3.25; AD14 0.25,-3.25; AD16 0.75,-3.25; AD18 1.25,-3.25; AD20 1.75,-3.25; AD22 2.25,-3.25; AD23 2.75,-3.25; B1 -3.25,2.75; B3 -2.5,2.75; B5 -2,2.75; B7 -1.5,2.75; B9 -1,2.75; B11 -0.5,2.75; B13 0,2.75; B15 0.5,2.75; B17 1,2.75; B19 1.5,2.75; B24 3.25,2.75; C1 -3.25,2.25; D2 -2.75,2; D23 2.75,2; E24 3.25,1.75; F2 -2.75,1.5; F23 2.75,1.5; G1 -3.25,1.25; H2 -2.75,1; H23 2.75,1; J1 -3.25,0.75; J24 3.25,0.75; K2 -2.75,0.5; L1 -3.25,0.25; L24 3.25,0.25; M2 -2.75,0; N1 -3.25,-0.25; N24 3.25,-0.25; P2 -2.75,-0.5; P23 2.75,-0.5; R1 -3.25,-0.75; R24 3.25,-0.75; T2 -2.75,-1; T23 2.75,-1; U1 -3.25,-1.25; U24 3.25,-1.25; V23 2.75,-1.5; W1 -3.25,-1.75; W24 3.25,-1.75; Y2 -2.75,-2; Y23 2.75,-2 | smd 4.85 x 4.85: GND 0,0
DFN-6/3MM = smd 0.85 x 0.45: 1 -1.45,1; 2 -1.45,0; 3 -1.45,-1; 4 1.45,-1; 5 1.45,0; 6 1.45,1 | smd 1.6 x 2.5: P$1 0,0
TXC-7V = smd 1.4 x 1.2: 1 -1.1,-0.85; 2 1.1,-0.85; 3 1.1,0.85; 4 -1.1,0.85
ABS05 = smd 0.5 x 1: A -0.55,0; B 0.55,0
2-SMD = smd 1.092 x 1.905: 1 -1.245,0; 2 1.245,0

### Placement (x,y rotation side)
A2  25.31,23.19 270 top
BT1  16,54.32 90 bottom
BT2  11.18,15.24 270 bottom
BT3  11.18,38.1 270 bottom
BT4  13.46,26.42 90 bottom
C1  18.73,23.33 180 top
C2  18.73,20.79 180 top
C3  11.68,22.86 90 top
C4  13.56,19.39 0 top
C5  19.05,10.67 90 top
C6  17.53,9.65 0 top
C7  7.87,29.97 0 top
C8  16.75,21.89 90 top
C9  24.89,55.34 0 top
C10  19.3,49.28 270 top
C11  14.06,14.95 90 top
C12  24.73,19.77 0 top
C13  25.15,16 270 top
C14  16.73,11.52 270 top
C15  15.21,19.27 90 top
C16  23.24,4.7 90 top
C17  16.76,2.29 0 top
C18  7.37,20.32 0 top
C19  7.37,21.34 0 top
C20  7.63,52.18 0 top
C21  15.72,11.52 270 top
C22  15.34,14.95 90 top
C23  22.23,4.7 90 top
C24  21.21,4.7 90 top
C25  7.62,28.7 0 top
C26  23.11,12.45 0 top
C27  18.29,49.28 270 top
C28  25.15,53.05 0 top
C29  16.89,44.45 180 top
C30  16.89,38.48 180 top
C31  16.51,1.02 0 top
C32  1.78,31.24 90 top
C33  7.37,31.24 90 top
D1  25.15,51.18 270 top
D2  10.41,15.49 0 top
J1  24.38,30.86 90 top
J5  5.5,60 180 top
L1  19.24,22.06 270 top
L2  13.3,13.93 270 top
L3  24.64,41.15 270 top
L4  14.83,13.42 0 top
L5  22.86,47.72 180 top
Q1  5.33,13.84 90 top
Q2  5.33,19.94 270 top
Q3  19.56,5.08 270 top
Q4  25.4,5.08 90 top
Q5  15.75,48.48 0 top
Q6  18.29,46.96 0 top
Q7  22.35,2.03 0 top
Q8  5.33,16.38 0 top
Q10  10.67,9.91 180 top
R1  11.68,12.7 270 top
R2  9.14,12.7 270 top
R3  10.41,12.7 270 top
R4  11.18,56.39 90 top
R5  10.41,51.82 270 top
R6  1.21,23.23 0 top
R7  2.98,23.23 180 top
R8  23.88,7.75 180 top
R9  21.34,6.6 0 top
R10  2.16,43.56 180 top
R11  2.03,28.96 90 top
R12  0.89,28.96 90 top
R13  16.89,41.27 0 top
R14  12.19,57.4 270 top
R15  12.7,52.83 90 top
R16  12.7,50.8 270 top
R17  12.19,55.37 90 top
R18  13.72,55.37 270 top
R19  11.43,50.8 90 top
R20  11.43,52.83 270 top
R21  13.72,57.4 90 top
R22  16.89,42.67 180 top
R23  23.88,6.6 180 top
R24  17.78,3.81 270 top
R25  7.11,18.54 180 top
R26  5.59,22.61 0 top
R27  11.43,8.38 180 top
S1  2.54,39.12 270 top
SJ1  20.19,57.63 0 top
SJ2  1.27,45.97 90 top
SJ3  5.33,43.94 90 top
SJ4  5.33,45.97 270 top
SJ5  3.3,45.97 270 top
TP1  1.02,9.91 0 bottom
TP2  1.02,25.15 0 top
TP3  21.59,11.43 0 top
TP4  1.02,9.91 0 top
TP5  14.73,4.83 0 top
TP6  7.87,27.18 0 top
TP7  15.75,5.59 0 top
TP8  7.87,17.27 0 top
TP9  23.62,1.02 0 bottom
TP10  20.32,5.84 0 bottom
TP11  15.49,8.64 0 top
TP12  5.59,17.78 0 bottom
TP13  10.16,23.88 0 top
TP14  10.03,21.46 0 top
TP15  6.6,23.62 0 bottom
TP16  1.02,26.16 0 top
TP17  23.11,35.05 0 bottom
TP18  25.27,12.57 0 top
TP19  14.99,1.78 0 top
TP20  25.4,10.92 0 bottom
TP21  22.1,7.87 0 top
TP22  9.4,0.76 0 top
TP23  23.62,51.31 0 top
TP24  9.4,19.3 0 top
TP25  21.34,38.61 0 top
TP26  26.16,59.18 0 top
TP27  26.16,57.91 0 top
U1  5.08,27.18 0 top
U2  20.07,53.05 90 top
U3  5.5,5.56 0 top
U4  3.56,50.47 90 top
U5  25.15,2.03 90 top
U6  12.95,1.78 270 top
U7  19.94,41.27 90 top
U8  19.81,2.29 90 top
U9  2.03,13.34 90 top
U10  19.99,16.61 90 top
U11  2.02,19.88 270 top
U$2  [UCB_CAL_200MIL]  6.86,39.12 0 top
X1  13.68,22.19 90 top
X3  18.03,11.18 90 top
X4  4.57,30.73 0 top

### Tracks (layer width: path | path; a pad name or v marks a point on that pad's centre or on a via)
!CLR_EN  (via drill 0.15, 0.2)
  Top 0.152: Q7.2 v21.34,2.03 | v25.4,4.06 Q4.2 | Q4.5 v25.4,6.1
  Top 0.254: R23.1 24.89,6.6 v25.4,6.1
  Bottom 0.152: v21.34,2.03 21.84,1.52 23.62,1.52 | 23.62,1.52 24.13,1.52 25.65,3.05 25.65,3.81 v25.4,4.06 v25.4,6.1 26.62,7.57 26.62,16.56 24.57,18.61 U10.AC21 | TP9.P$1 23.62,1.52
  other vias: 22.74,18.61
!CLR_INT  (via drill 0.15, 0.2)
  Top 0.152: U5.5 v25.15,3.5
  Top 0.203: v25.15,7.62 25.02,7.75 R8.1
  Bottom 0.152: v25.15,3.5 24.69,3.5 24.38,3.81 24.38,6.86 v25.15,7.62 26.31,8.79 26.31,10.92 | U10.AC19 24.64,18.11 26.31,16.43 26.31,10.92 | TP20.P$1 26.31,10.92
  other vias: 22.74,18.11
!FTDI_RESET  (via drill 0.2)
  Top 0.203: U4.18 4.81,53.54 v4.83,53.56 | v4.32,44.45 5.24,44.45 SJ3.2
  Bottom 0.203: v4.83,53.56 4.32,53.05 v4.32,44.45
!HUM_EN  (via drill 0.2)
  Top 0.152: U10.A20 16.67,18.29 16.62,18.34 14.33,18.34 14.12,18.54 v13.72,18.54
  Top 0.203: Q2.5 v5.33,18.92 | Q8.5 v6.35,16.38 | Q2.2 v5.33,21.59 5.33,22.43 R26.1
  Route2 0.152: v13.72,18.54 8.89,18.54 5.84,21.59 v5.33,21.59
  Bottom 0.152: TP12.P$1 6.35,17.78
  Bottom 0.203: v5.33,21.59 5.33,19.05 | 5.33,19.05 v5.33,18.92 | 5.33,19.05 6.35,18.03 6.35,17.78 v6.35,16.38
!LT_EN  (via drill 0.2)
  Top 0.152: Q3.5 19.56,3.89 v19.48,3.81 | Q7.5 v23.37,2.03 | Q3.2 v19.56,6.1 | R24.1 17.78,4.83 19.05,6.1 v19.56,6.1 | U10.AD20 25.33,18.36 26.31,17.37 26.31,12.27 22.73,8.69 21.54,8.69 19.63,6.78 19.63,6.17 v19.56,6.1
  Bottom 0.152: v19.48,3.81 19.56,3.81 | 19.56,3.81 21.59,3.81 v23.37,2.03 | 19.56,3.81 v19.56,6.1 20.07,6.1 TP10.P$1
!LT_INT
  Top 0.152: 20.57,4.06 20.57,6.28 R9.1 22.1,7.8 TP21.P$1 22.35,7.87 26.62,12.14 26.62,17.53 25.29,18.86 U10.AD22
  Top 0.203: U8.4 20.57,3.32 20.57,4.06 | R9.1 20.83,6.68
!PIR_EN  (via drill 0.2)
  Top 0.152: U10.AD12 23.77,16.36 24.27,15.86 24.27,15.5 24.27,15.49 24.27,12.3 21.87,9.91 21.29,9.91 | 11.86,9.14 15.49,9.14 | 15.49,9.14 20.27,9.14 21.03,9.91 21.29,9.91 | TP11.P$1 15.49,9.14 | 21.29,9.91
  Top 0.203: Q10.2 11.53,9.91 v11.86,9.58 11.86,9.14 R27.1
!PR_EN  (via drill 0.15 pad 0.3, 0.2)
  Top 0.152: v6.86,17.78 7.37,17.27 TP8.P$1
  Top 0.203: Q1.5 v5.33,14.86 | Q1.2 v5.33,12.83 | Q8.2 4.32,16.38 v4.06,16.64 3.81,16.89 3.81,17.53 4.06,17.78 5.84,17.78 v6.86,17.78 7.54,18.47 R25.1
  Route2 0.152: U10.B19 7.19,18.11 v6.86,17.78
  Bottom 0.203: v5.33,12.83 v5.33,14.86 4.06,16.13 v4.06,16.64
  other vias: 17.24,18.11
!RST  (via drill 0.15, 0.2)
  Top 0.152: v25.91,30.73 25.78,30.86 J1.3 | U1.1 2.63,27.93 R11.1 2.62,28.52 v2.79,28.7
  Top 0.203: SJ3.1 5.59,43.29 v5.59,42.67
  Route15 0.152: U10.AC13 23.37,17.24 23.37,19.81 22.86,20.32 20.83,20.32 20.57,20.57 20.57,28.19 23.11,30.73 v25.91,30.73
  Bottom 0.152: v2.79,28.7 4.83,30.73 5.59,30.73 | 5.59,30.73 21.84,30.73 | 21.84,30.73 v25.91,30.73 | v5.59,42.67 5.59,30.73 | TP17.P$1 21.84,33.78 21.84,30.73
  other vias: 22.74,16.61
!RTC_EXTR  (via drill 0.2)
  Top 0.152: U1.3 v2.8,26.93 v2.79,26.92
  Top 0.203: 3.45,36.49 S1.P$4 | S1.P$4 S1.P$2 3.45,42.7 R10.1 | v3.3,34.8 3.45,34.94 S1.P$4
  Bottom 0.203: v2.79,26.92 2.29,27.43 2.29,33.78 v3.3,34.8
!RTC_IRQ1
  Top 0.152: U1.11 6.58,27.28 6.88,27.28 7.11,27.04 7.11,25.91 9.65,23.37 | 9.65,23.37 11.18,21.84 11.18,20.32 13.46,18.03 16.04,18.03 16.71,17.36 U10.A16 | TP13.P$1 9.65,23.37
!RTC_IRQ2  (via drill 0.15, 0.2)
  Top 0.152: U1.4 3.68,24.82 4.67,23.82 7.92,23.82 v9.65,22.1 10.03,21.72 TP14.P$1
  Bottom 0.152: v9.65,22.1 11.94,22.1 16.93,17.11 U10.B15
  other vias: 17.24,17.11
!RTC_IRQ3  (via drill 0.2)
  Top 0.152: U1.8 5.83,25.41 v6.6,24.64 7.11,24.13 8.38,24.13 10.67,21.84 10.67,20.32 13.26,17.73 15.84,17.73 16.71,16.86 U10.A14
  Bottom 0.152: 5.84,25.4 v6.6,24.64 TP15.P$1
!VBAT_PRI_ON  (via drill 0.2)
  Top 0.203: Q6.2 v17.27,46.96 | Q6.5 v19.3,46.96 | U2.10 19,54.86
  Top 0.406: 19,54.86 v17.78,54.86
  Bottom 0.203: v17.27,46.96 v19.3,46.96
  Bottom 0.61: v17.78,54.86 17.53,54.61 17.53,47.21 v17.27,46.96
!VBAT_SEC_ON  (via drill 0.2)
  Top 0.203: Q5.2 v14.73,48.48 | Q5.5 v16.76,48.48
  Top 0.406: U2.9 v19.57,55.87 v19.56,55.88
  Bottom 0.203: v14.73,48.48 v16.76,48.48
  Bottom 0.61: v19.56,55.88 17.72,55.88 16.54,54.7 16.54,54.21 16.51,54.18 16.51,54.1 14.73,52.32 v14.73,48.48
ACC_CS  (via drill 0.15, 0.2)
  Top 0.152: U6.2 13.3,2.62 13.3,2.81 14.3,3.81 15.37,3.81 16.19,4.63 | 16.19,4.63 21.16,9.6 22.1,9.6 24.64,12.14 24.64,13.08 v24.77,13.21 | 16.19,4.63 15.75,5.08 TP7.P$1
  Bottom 0.152: v24.77,13.21 24.71,13.26 24.71,15.93 23.03,17.61 U10.AC17 22.78,17.61
  other vias: 22.74,17.61
ACC_INT1
  Top 0.152: U6.12 14.02,2.03 21.29,9.3 22.35,9.3 25.32,12.27 | U10.AD16 25.39,17.36 25.65,17.09 25.65,12.6 25.32,12.27 | TP18.P$1 25.27,12.32 25.32,12.27
ACC_INT2
  Top 0.152: U6.11 13.8,1.62 14.04,1.62 14.59,2.17 | 14.59,2.17 21.41,8.99 22.61,8.99 26.01,12.39 26.01,17.17 25.32,17.86 U10.AD18 | TP19.P$1 14.59,2.17
D+
  Top 0.203: J5.3 5.5,54.67 5.84,54.32 7.62,54.32 9.14,52.8 9.14,51.53 8.64,51.02 6.33,51.02 6.14,51.22 U4.14
D-
  Top 0.203: U4.15 6.67,51.72 6.86,51.53 8.38,51.53 8.64,51.78 8.64,52.55 7.37,53.82 5.33,53.82 4.85,54.3 J5.2
DBG_RX  (via drill 0.2)
  Top 0.152: U10.G1 18.74,12.27 v18.81,12.2
  Top 0.203: SJ5.2 3.3,43.94 v15.75,31.5
  Route2 0.152: v18.81,12.2 18.81,13.45 17.78,14.48 17.78,18.29 15.75,20.32 v15.75,31.5
DBG_TX  (via drill 0.15, 0.2)
  Top 0.203: SJ4.2 5.49,45.56 v16.26,34.8
  Route2 0.152: U10.H2 18.09,14.77 18.09,18.41 16.26,20.24 v16.26,34.8
  other vias: 18.99,13.86
FTDI_VCCIO
  Top 0.203: U4.1 1.81,46.92 SJ2.2
GND  (via drill 0.2, 0.25, 0.41)
  Top 0.102: 18.53,18.64 18.53,18.63 | U10.F23 18.49,19.57 18.62,19.7 18.62,20.47 C2.2
  Top 0.152: U8.2 19.81,0.81 21.34,0.81 v21.34,1.27
  Top 0.203: C20.2 8.06,52.36 7.37,53.05 | C1.2 17.84,23.33 | U10.B7 17.9,15.11 | 17.9,15.11 18.03,15.24 | U10.GND 18.49,15.11 17.9,15.11 | U10.F23 18.49,18.54 | 18.49,18.54 18.49,18.14 v18.59,18.03 | U10.GND 19.99,17.04 18.49,18.54 | U10.GND 19.99,17.18 18.53,18.64 | U4.4 3.31,47.85 3.56,47.6 4.97,47.6 5.08,47.5 5.59,47.5
  Top 0.254: U6.8 12.7,0.51 12.19,0.51 12.2,0.52 U6.7 12.19,1.02 11.68,1.02 11.68,1.52 | 11.68,1.52 11.69,1.53 U6.6 | 11.68,1.52 11.68,2.03 U6.5 | C4.1 12.7,19.81 v12.45,19.81 | v17.53,23.62 17.82,23.33 C1.2 | U8.EP C17.2
  Top 0.406: U9.4 1.03,15.13 1.27,15.37 4.57,15.37
  other vias: 18.29,51.28 6.35,53.31 8.89,54.07 11.94,51.78 12.95,56.36 4.57,14.86 21.84,42.16 21.84,40.39 19.3,53.85 20.07,53.85 20.83,53.85 20.83,53.09 20.07,53.09 19.3,53.09 19.3,52.32 20.07,52.32 20.83,52.32 1.78,54.07 22.1,50.26 19.99,18.03 19.99,16.61 19.99,15.16 18.59,16.61 21.41,16.61 21.41,15.16 21.41,18.03 18.59,15.16 14.48,24.38 14.48,18.8 5.08,27.18 23.11,13.21 4.7,27.56 5.46,27.56 5.46,26.8 4.7,26.8 19.81,46.1 9.14,20.07 21.34,5.84 17.53,20.83 17.53,21.59 17.53,22.61 17.91,24.26 21.08,22.61 21.08,21.72 21.08,20.83 22.35,20.83 23.62,20.83 24.89,20.83 26.16,20.83 21.08,23.62 21.08,25.15 21.08,26.42 18.54,24.38 22.35,26.42 23.62,26.42 24.89,26.42 26.16,26.42 25.15,13.72 17.02,10.41 18.8,9.6 19.18,24.77 20.07,25.15 2.03,22.61 18.03,1.27 25.4,7.11 23.37,3.05 25.4,0.51 20.07,23.62 20.07,22.61 20.07,21.59 20.07,26.42 18.8,26.42 17.53,26.42 17.53,25.4 18.8,25.4 26.16,19.81 26.16,18.8 17.53,27.69 18.8,27.69 20.07,27.69 22.35,27.69 23.62,27.43 24.89,27.43 26.16,27.69
  pour Top (rank 2): 0,60 27,60 27,0 0,0
  pour Bottom (rank 2): 0,60 27,60 27,0 0,0
  pour Top (rank 2, no thermals): 24.55,22.05 26.07,22.05 26.07,20.76 24.55,20.76
  pour Route2 (rank 2): 0,60 0,0 27,0 27,60
LBST
  Top 0.254: U2.20 21.07,49.51 21.08,50.01
  Top 0.406: 21.08,50.01 21.08,47.79 L5.P$1
LED_BLUE  (via drill 0.15, 0.2)
  Top 0.203: R3.2 10.59,12.27 v11.18,11.68
  Bottom 0.203: v11.18,11.68 19.05,11.68 19.81,12.45 19.81,12.7 19.81,13.54 U10.K2
  other vias: 19.49,13.86
LED_GREEN  (via drill 0.2)
  Top 0.152: U10.L1 19.74,11.61 v19.68,11.56
  Top 0.203: v9.14,11.18 R2.2
  Bottom 0.203: v9.14,11.18 19.3,11.18 v19.68,11.56
LED_RED  (via drill 0.2)
  Top 0.152: U10.J1 19.24,12.76 v19.3,12.7
  Top 0.203: R1.2 11.76,12.19 v13.46,12.19
  Bottom 0.203: v13.46,12.19 17.02,12.19 17.53,12.7 v19.3,12.7
MISO  (via drill 0.2)
  Top 0.152: U6.3 v12.7,3.17 | v20.78,10.41 20.78,13.32 U10.R1 | U1.6 4.83,24.89 v5.08,24.64 | v7.37,5.08 3.81,5.08 1.02,7.87 TP4.P$1
  Route15 0.152: v5.08,24.64 7.62,22.1 7.62,5.33 v7.37,5.08
  Bottom 0.152: v20.78,10.41 20.78,9.19 15.15,3.57 14.21,3.57 13.81,3.17 v12.7,3.17 9.27,3.17 v7.37,5.08
MOSI  (via drill 0.2)
  Top 0.152: 12.27,2.59 U6.4 12.2,3.29 12.19,3.3 12.57,3.68 v13.34,3.68 14.48,4.83 TP5.P$1 | v20.22,9.91 20.22,13.34 U10.N1 | U1.9 6.43,25.57 v7.37,24.64
  Route15 0.152: v13.34,3.68 9.02,3.68 8.23,4.47 8.23,23.77 v7.37,24.64
  Bottom 0.152: v13.34,3.68 13.53,3.87 14.99,3.87 20.22,9.11 v20.22,9.91
N$1
  Top 0.254: SJ1.3 21.84,57.75 21.84,58.39 21.08,59.15 12.41,59.15 11.18,57.91 R4.2 12.04,56.82 R14.2
N$2
  Top 0.152: C14.1 17.74,12.96 U10.C1
N$3  (via drill 0.15, 0.2)
  Top 0.203: U10.E24 18.23,19.87 18.2,19.87
  Top 0.254: L2.1 13.45,14.51 C11.1 C22.1 15.43,14.61 v16.51,14.61 U10.B5
  Bottom 0.406: U10.E24 17.78,19.4 17.78,15.11 17.27,14.61 v16.51,14.61
  other vias: 18.24,19.86
N$4
  Top 0.152: 16.75,21.13 16.75,21.43 C8.1
  Top 0.203: U10.D23 17.65,19.71 17.65,20.03 16.75,20.93 16.75,21.43
N$5
  Top 0.102: U10.H23 18.99,19.61 18.89,19.71 18.89,20.52 C2.1
  Top 0.305: 19.24,20.87 C2.1 19.16,21.55 arc-90 L1.2
N$6
  Top 0.305: 25.33,24.5 A2.S1 20.35,24.52 arc90 C1.1 19.16,22.57 arc90 L1.1
N$7
  cutout Route2: 21.24,21.02 26.96,21.02 26.96,26.1 21.24,26.1
N$8
  Top 0.203: C3.2 X1.3 12.83,24.01 13.66,24.84 14.67,24.84 15.39,24.12 15.39,21.71 15.88,21.22 U10.B24
N$9
  Top 0.203: C4.2 13.99,20.54 X1.1 15.05,21.09 15.05,21.06 U10.A23
N$10
  cutout Top: 0,22.48 1.78,22.48 1.78,20.95 2.29,20.95 2.29,22.48 4.32,22.48 4.32,10.79 0,10.79
N$11
  cutout Top: 19.68,19.3 17.91,19.3 17.91,23.88 19.68,23.88
N$12
  Top 0.203: R13.2 20.19,41.27 20.59,41.67 U7.4
N$13
  Top 0.203: U4.16 7.16,52.22 C20.1
N$14
  Top 0.203: U7.6 18.81,42.67 R22.1
N$15
  Top 0.203: D2.2 11.68,14.22 R1.1
N$16  (via drill 0.2)
  Top 0.254: SJ1.1 18.26,57.63 14.22,53.59 v14.22,53.31 | R5.2 10.56,51.23 10.67,51.23 | 10.67,51.23 R19.2 | v10.67,50.55 10.67,51.23
  Bottom 0.254: v10.67,50.55 11.46,50.55 v14.22,53.31
N$17
  Top 0.203: D2.4 9.14,15.09 R2.1
N$18  (via drill 0.2)
  Top 0.254: R19.1 R16.2 13.03,50.34 13.46,50.77 13.46,53.56 14.73,54.83 14.73,58.42 | U2.7 20.57,54.8 v20.57,55.85 | R14.1 R21.2 14.3,58.42 14.73,58.42 | 14.73,58.42 v17.02,58.42
  Bottom 0.254: v17.02,58.42 18.03,58.42 20.57,55.88 v20.57,55.85
N$19
  Top 0.203: D2.3 9.98,13.56 R3.1
N$20
  Top 0.152: U8.1 19.16,0.65 19.3,0.51 21.59,0.51 21.93,0.84 Q7.3
N$21
  Top 0.203: Q8.6 5.92,16.89 6.6,16.89 7.11,16.38
  Top 0.406: 7.11,16.38 7.11,13.08 5.33,11.3 1.27,11.3 1.02,11.56 1.02,12.32 U9.1
N$22
  Top 0.152: Q8.3 3.4,16.03
  Top 0.406: 3.4,16.03 2.02,17.41 U11.5
N$23
  Top 0.203: Q10.6 5.9,9.56 U3.VCC
N$25
  Top 0.203: U1.14 5.33,29.21 5.59,29.46 6.93,29.46 C7.1
N$26
  Top 0.203: U1.16 4.33,29.2 3.33,30.2 X4.1 1.85,30.73 C32.1
N$27
  Top 0.203: U1.15 4.83,29.21 5.59,29.97 5.84,29.97 5.82,30 X4.2 7.29,30.73 C33.1
N$31
  Top 0.152: Q7.6 22.93,2.54 23.54,2.54 U5.1
N$32
  Top 0.254: U2.8 20.07,57.5 SJ1.2
N$34
  Top 0.152: Q1.6
  Top 0.203: U9.3 3.1,14.27 Q1.6
N$35
  cutout Route15: 21.24,21.02 26.96,21.02 26.96,26.1 21.24,26.1
N$38
  cutout Top: 21.24,26.1 26.96,26.1 26.96,23.32 26.96,21.02 26.07,21.02 26.07,22.05 24.55,22.05 24.55,21.02 21.24,21.02
N$39
  cutout Bottom: 21.24,21.02 26.96,21.02 26.96,26.1 21.24,26.1
N$41
  Top 0.203: U9.2 5.6,12.34 5.84,12.57 5.84,13.26 Q1.3
  Top 0.254: 3.05,12.32 U9.2
N$44
  Top 0.254: L4.2 16.57,13.42 16.57,13.44 U10.B3
N$45
  Top 0.203: Q5.1 15.16,48.99 14.48,48.99 14.22,48.74 14.22,47.47 14.48,47.21 16,47.21 16.17,47.38 Q5.4
N$48
  Top 0.152: Q2.3
  Top 0.203: U11.1 4.02,21.32 Q2.3
N$49
  Top 0.254: L4.1 13.38,13.42 L2.2
N$50
  Top 0.152: Q2.6
  Top 0.203: U11.6 3.03,18.41 5.59,18.41 5.84,18.67 5.84,19.36 Q2.6
N$51
  Top 0.152: U8.6 19.14,3.21 18.54,3.81 18.54,5.08 18.97,5.5 Q3.3
N$52
  Top 0.152: Q3.6 19.91,3.31 U8.5
N$53
  Top 0.152: Q6.4
  Top 0.203: Q6.1 17.7,47.47 17.02,47.47 16.76,47.21 16.76,46.03 17.06,45.73 18.33,45.73 18.71,46.11 Q6.4
N$54
  Top 0.152: Q4.3 25.9,4.5 25.9,2.96 U5.4
N$55
  Top 0.152: Q4.6 24.9,5.36 24.38,4.84 24.38,2.97 U5.6
N$57  (via drill 0.2)
  Top 0.254: U2.12 15.79,53.55 v15.37,53.98 | R17.1 12.27,54.86 12.7,54.86 | 12.7,54.86 v12.95,54.86 13.64,54.86 R18.2 | 12.7,54.86 R15.2 R20.1
  Bottom 0.254: v15.37,53.98 14.48,54.86 v12.95,54.86
N$58  (via drill 0.2)
  Top 0.254: 11.41,52.34 R20.2 11.28,52.25 R5.1 v10.41,55.37 11,55.95 R4.1 12.09,55.95 12.19,55.85 R17.2 | U2.11 16.3,54.05 v15.88,54.48
  Bottom 0.254: v15.88,54.48 14.99,55.37 v10.41,55.37
PIR_OUT  (via drill 0.15)
  Top 0.152: U3.OUT 6.65,0.81 9.35,0.81 TP22.P$1
  Bottom 0.152: U3.OUT 5.18,2.29 14.73,2.29 24.3,11.85 24.3,15.91 24.1,16.11 U10.AC11
  other vias: 22.74,16.11
RTC_CS  (via drill 0.15, 0.2)
  Top 0.152: U1.12 6.44,27.94 v7.37,27.94 | 7.87,27.43 TP6.P$1
  Top 0.203: v7.37,27.94 7.87,27.43
  Bottom 0.152: v7.37,27.94 8.38,28.96 10.16,28.96 10.92,28.19 10.92,23.55 16.86,17.61 U10.B17
  other vias: 17.24,17.61
RXD
  Top 0.203: U4.2 2.31,47.73 2.79,47.24 4.83,47.24 5.33,46.74 SJ4.1
SCK  (via drill 0.2)
  Top 0.152: U6.1 13.78,2.53 v14.39,3.14 | v21.34,10.41 21.24,10.51 21.24,11.43 | 21.24,11.43 U10.U1 | U1.7 5.33,25.15 v5.84,24.64 | TP3.P$1 21.24,11.43
  Route15 0.152: v5.84,24.64 7.92,22.55 7.92,4.27 9.65,2.54 13.79,2.54 v14.39,3.14
  Bottom 0.152: v14.39,3.14 15.15,3.14 21.25,9.23 21.25,10.32 v21.34,10.41
SCL  (via drill 0.15, 0.2)
  Top 0.152: Q4.1 24.84,4.45 v24.84,4.06 | Q2.1 6.14,20.36 v6.22,20.45 | TP2.P$1 1.02,24.38 v0.76,24.13
  Top 0.203: Q1.1 4.57,13.01 v4.57,12.83 | v0.76,24.13 0.76,23.24 R6.1 | Q3.1 20.07,5.66 v20.07,6.6
  Route2 0.152: v4.57,12.83 11.3,6.1 18.8,6.1 19.3,6.6 v20.07,6.6 | U10.AC9 22.35,15.22 22.35,6.66 22.3,6.6
  Route2 0.203: v4.57,12.83 4.06,13.34 4.06,14.99 4.12,15.04 4.12,15.05 6.22,17.16 v6.22,20.45 | v24.84,4.06 22.3,6.6 v20.07,6.6
  Bottom 0.203: v0.76,24.13 1.02,24.38 4.32,24.38 6.1,22.61 6.1,20.57 v6.22,20.45 | v20.07,6.6 20.32,6.86
  other vias: 22.74,15.61
SDA  (via drill 0.2)
  Top 0.152: 3.56,23.09 R7.1 | Q3.4 19,4.44 v19,4.12 | Q4.4 26.34,6.1 v26.42,6.1 | v23.84,15.68 23.66,15.86 U10.AD10
  Top 0.203: Q2.4 4.65,19.18 v4.32,19.18 | Q1.4 6.02,14.61 v6.35,14.61 | R7.1 3.95,23.23 v4.06,23.11
  Route2 0.152: v6.35,2.79 12.34,2.79 12.52,2.62 17.49,2.62 v19,4.12 | v23.84,15.68 26.42,13.11 v26.42,6.1
  Route2 0.203: v19,4.12 19.14,4.12 19.29,4.27 20.38,4.27 21.79,2.86 21.79,2.85 23.11,1.52 25.65,1.52 26.42,2.29 v26.42,6.1
  Bottom 0.152: v6.35,14.61 6.35,9.91 | 6.35,9.91 v6.35,2.79 | TP1.P$1 6.35,9.91
  Bottom 0.203: v6.35,14.61 4.83,16.13 4.83,18.92 4.57,19.18 v4.32,19.18 4.32,22.86 v4.06,23.11
SW  (via drill 0.15, 0.2)
  Route15 0.152: U10.B11 16.76,16.59 16.76,35.05 v20.32,38.61
  other vias: 17.24,16.11
  pour Top (isolate 0.203, no thermals): 19.81,40.77 19.81,37.85 26.16,37.85 26.16,39.5 20.07,39.5 20.07,40.77
SWDCLK  (via drill 0.15, 0.2)
  Top 0.152: J1.4 22.59,29.7 v22.59,29.48
  Bottom 0.152: U10.AA24 20.78,19.86 19.63,21.01 19.63,26.52 v22.59,29.48
  other vias: 22.24,19.86
SWDIO  (via drill 0.15, 0.2)
  Top 0.152: v22.86,28.96 23.5,29.59 J1.2
  Bottom 0.152: U10.AC24 22.74,20.18 22.61,20.32 20.83,20.32 20.57,20.57 20.57,26.67 v22.86,28.96
  other vias: 22.74,19.86
TXD  (via drill 0.2)
  Top 0.203: U4.30 0.69,49.72 0.51,49.53 v0.51,47.75 | v2.29,46.74 2.94,46.74 SJ5.1
  Bottom 0.203: v0.51,47.75 1.52,46.74 v2.29,46.74
USB_5V
  Top 0.203: U4.19 4.31,55.77 J5.1
VBAT  (via drill 0.2)
  Top 0.152: Q6.6 18.71,47.47 | U1.5 4.33,24.9 v4.32,24.89 | v14.56,16.85 15.72,16.85 16.54,16.03 16.59,15.98 16.71,15.86 U10.A10
  Top 0.254: v18.8,47.97 18.71,47.89 18.71,47.47 18.71,47.34 | U2.14 17.3,52.55 17.27,52.58
  Top 0.508: BT3.POS2 12.78,49.33 13.99,50.55 13.99,52.09 14.92,53.02 16.57,53.02 17.02,52.58 17.27,52.58
  Route15 0.254: BT2.POS1 9.18,25.15 4.57,25.15 v4.32,24.89
  Route15 0.406: v18.8,47.97 17.24,47.97 14.67,45.4 BT4.+
  pour Route15: 8.64,49.53 14.73,49.53 14.73,9.65 10.92,9.65 10.92,5.84 13.72,5.84 13.72,3.81 8.64,3.81
VCC  (via drill 0.2, 0.41)
  Top 0.152: U10.W1 21.74,13.61 21.75,13.62 | Q7.4 22.78,1.31 v22.48,1.02 | Q7.1 21.64,2.67 v21.34,2.67 | TP26.P$1 v25.4,58.42
  Top 0.203: C12.1 23.56,19.78 23.28,19.5 23.28,19.4 U10.AD23 | 15.22,18.85 C15.1 15.17,18.8 | 16.75,18.85 U10.A22 16.73,18.85 | Q8.1 4.73,16.73 v4.32,17.14 | 7.37,28.7 C25.1 7.11,28.7 5.95,28.7 U1.13 | R11.2 2,29.4 | 2,29.4 1.85,29.46 | Q10.1 11.09,8.48 11.09,8.47 | 11.09,8.47 R27.2 10.92,8.38 | C19.1 C18.1 6.68,20.07 6.68,19.3 | R25.2 6.68,19.3 | R6.2 2.03,23.23 | 2.03,23.23 R7.2 | 2.03,23.23 v2.03,23.88 | R10.2 1.78,43.61 v1.78,44.45 1.78,45.06 SJ2.1 | 6.68,19.3 v7.11,19.3 | v11.68,7.37 11.09,7.96 11.09,8.47 | U10.Y2 21.96,13.83 | R23.2 R8.2 | 15.85,1.03 C31.1 | U6.9 13.21,0.51 13.72,0.51 13.7,0.52 U6.10 | 25.15,16.26 C13.1 | Q8.4 6.3,15.49 v6.35,15.49 | R12.2 2,29.4 | D2.1 10.26,16.51 9.75,16.51 7.87,14.63 7.87,12.7 v7.11,11.94
  Top 0.254: 16.82,12.92 16.82,12.94 U10.B1 | U10.Y2 22.03,13.82 | v21.34,2.67 21.21,2.79 C24.1 C23.1 C16.1 23.57,4.27 23.88,4.57 23.88,5.84 23.44,6.28 R23.2 22.86,6.6 | R9.2 22.86,6.6 | U6.10 v14.72,1.03 | v14.72,1.03 14.74,1.03 | 14.74,1.03 15.85,1.03 | C31.1 15.86,1.81 C17.1 16.33,2.62 17.09,3.38 R24.2 | 14.74,1.03 v14.73,1.02 v14.72,1.03 | v22.86,7.11 22.86,6.6 | U10.A22 16,18.86 | 16,18.86 15.24,18.86 15.22,18.85 | R26.2 6.1,22.61 v6.6,22.1 6.93,21.77 C19.1 | J1.1 v26.16,28.45 | v16,19.43 16,18.86 | 7.11,28.7 7.12,28.7 7.75,29.33 v7.87,29.33 | R12.2 1.02,29.52 v1.02,30.23 | U10.AD14 v24.54,16.87 24.97,16.43 C13.1
  Top 0.305: 16.82,12.92 16.57,12.92 v16.32,12.66
  Top 0.406: 21.96,13.83 21.75,13.62 21.75,12.8 v21.84,12.7 22.1,12.45 C26.1 | C21.1 15.72,12.06 v16.32,12.66 | C12.1 v23.75,20.32
  other vias: 18.03,39.62 18.54,38.35
  pour Top (isolate 0.203, no thermals): 18.41,40.64 19.3,40.64 19.3,37.85 17.4,37.85 17.4,40.13 18.41,40.13
  pour Route15 (rank 2): 0,60 27,60 27,0 0,0
VOC_SAMP_VSTOR  (via drill 0.2)
  Top 0.152: C10.1 19.99,49.71
  Top 0.203: v20.57,50.29 20.57,50.52 U2.19 | Q5.6 17.05,49.71 C27.1
  Top 0.254: U2.3 21.82,53.07 23.31,53.07 23.35,53.11 v23.45,53.11 | C27.1 19.99,49.71 v20.57,50.29
  Bottom 0.406: v20.57,50.29 23.39,53.11 v23.45,53.11
VREF_SAMP
  Top 0.406: U2.4 22.61,53.55 24.39,55.34 C9.1
VSEC  (via drill 0.2)
  Top 0.152: U10.A8 16.64,15.36 15.9,16.11 13.51,16.11 10.31,19.3 v10.16,19.3 TP24.P$1
  Top 0.203: U2.18 20.07,50.77 19.81,50.51
  Top 0.406: 19.81,50.51 17.31,50.51 BT1.+
  Route2 0.152: v10.16,19.3 10.16,23.11 10.92,23.88 10.92,48.77 13.98,51.82 BT1.+
VSOL  (via drill 0.15)
  Top 0.406: U2.2 24.12,52.55 24.13,52.55
  Route15 0.152: D1.+ 23.88,49.91 23.88,41.4 17.07,34.59 17.07,20.52 17.78,19.81 17.78,16.07 17.32,15.61 U10.B9
  other vias: 17.24,15.61
  pour Top (no thermals): 23.88,53.56 23.88,52.55 22.86,51.53 22.86,46.2 26.16,46.2 26.16,51.28 24.89,52.55 24.89,53.56
VSW  (via drill 0.2, 0.41)
  Top 0.152: Q5.3
  Top 0.203: v14.73,47.72 14.91,47.72 Q5.3 | Q6.3 17.45,46.2 v17.27,46.2
  Top 0.305: R22.2 16.24,43.15 C29.1
  Bottom 0.61: v14.73,47.72 16.26,46.2 v17.27,46.2 18.8,44.67 v18.8,44.45
  pour Top (isolate 0.203, no thermals): 19.81,41.78 19.81,43.31 17.53,43.31 17.53,44.7 26.16,44.7 26.16,42.8 20.07,42.8 20.07,41.78
WDI
  Top 0.152: U1.2 2.29,27.43 | 2.29,27.43 1.98,27.43 R12.1 | 2.29,27.43 2.29,26.16 | 2.29,26.16 2.29,25.7 4.37,23.62 4.45,23.62 4.55,23.52 6.96,23.52 13.08,17.4 15.67,17.4 16.71,16.36 U10.A12 | TP16.P$1 2.29,26.16
XL1
  Top 0.102: U10.D2 17.99,13.61 18.09,13.51 18.09,12.82 17.33,12.06 17.33,11.33 X3.A
  Top 0.203: X3.A 17.96,10.55 C6.2
XL2
  Top 0.102: U10.F2 18.49,13.61 18.39,13.51 18.39,12.08 X3.B
  Top 0.203: C5.2 18.43,11.73 X3.B

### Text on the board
tNames: Other | Titanate | RESET | Permamote / Neal Jackson / 1/18

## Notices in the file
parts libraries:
SparkFun-Passives: Licensing: CC v3.0 Share-Alike You are welcome to use this library for commercial purposes.
